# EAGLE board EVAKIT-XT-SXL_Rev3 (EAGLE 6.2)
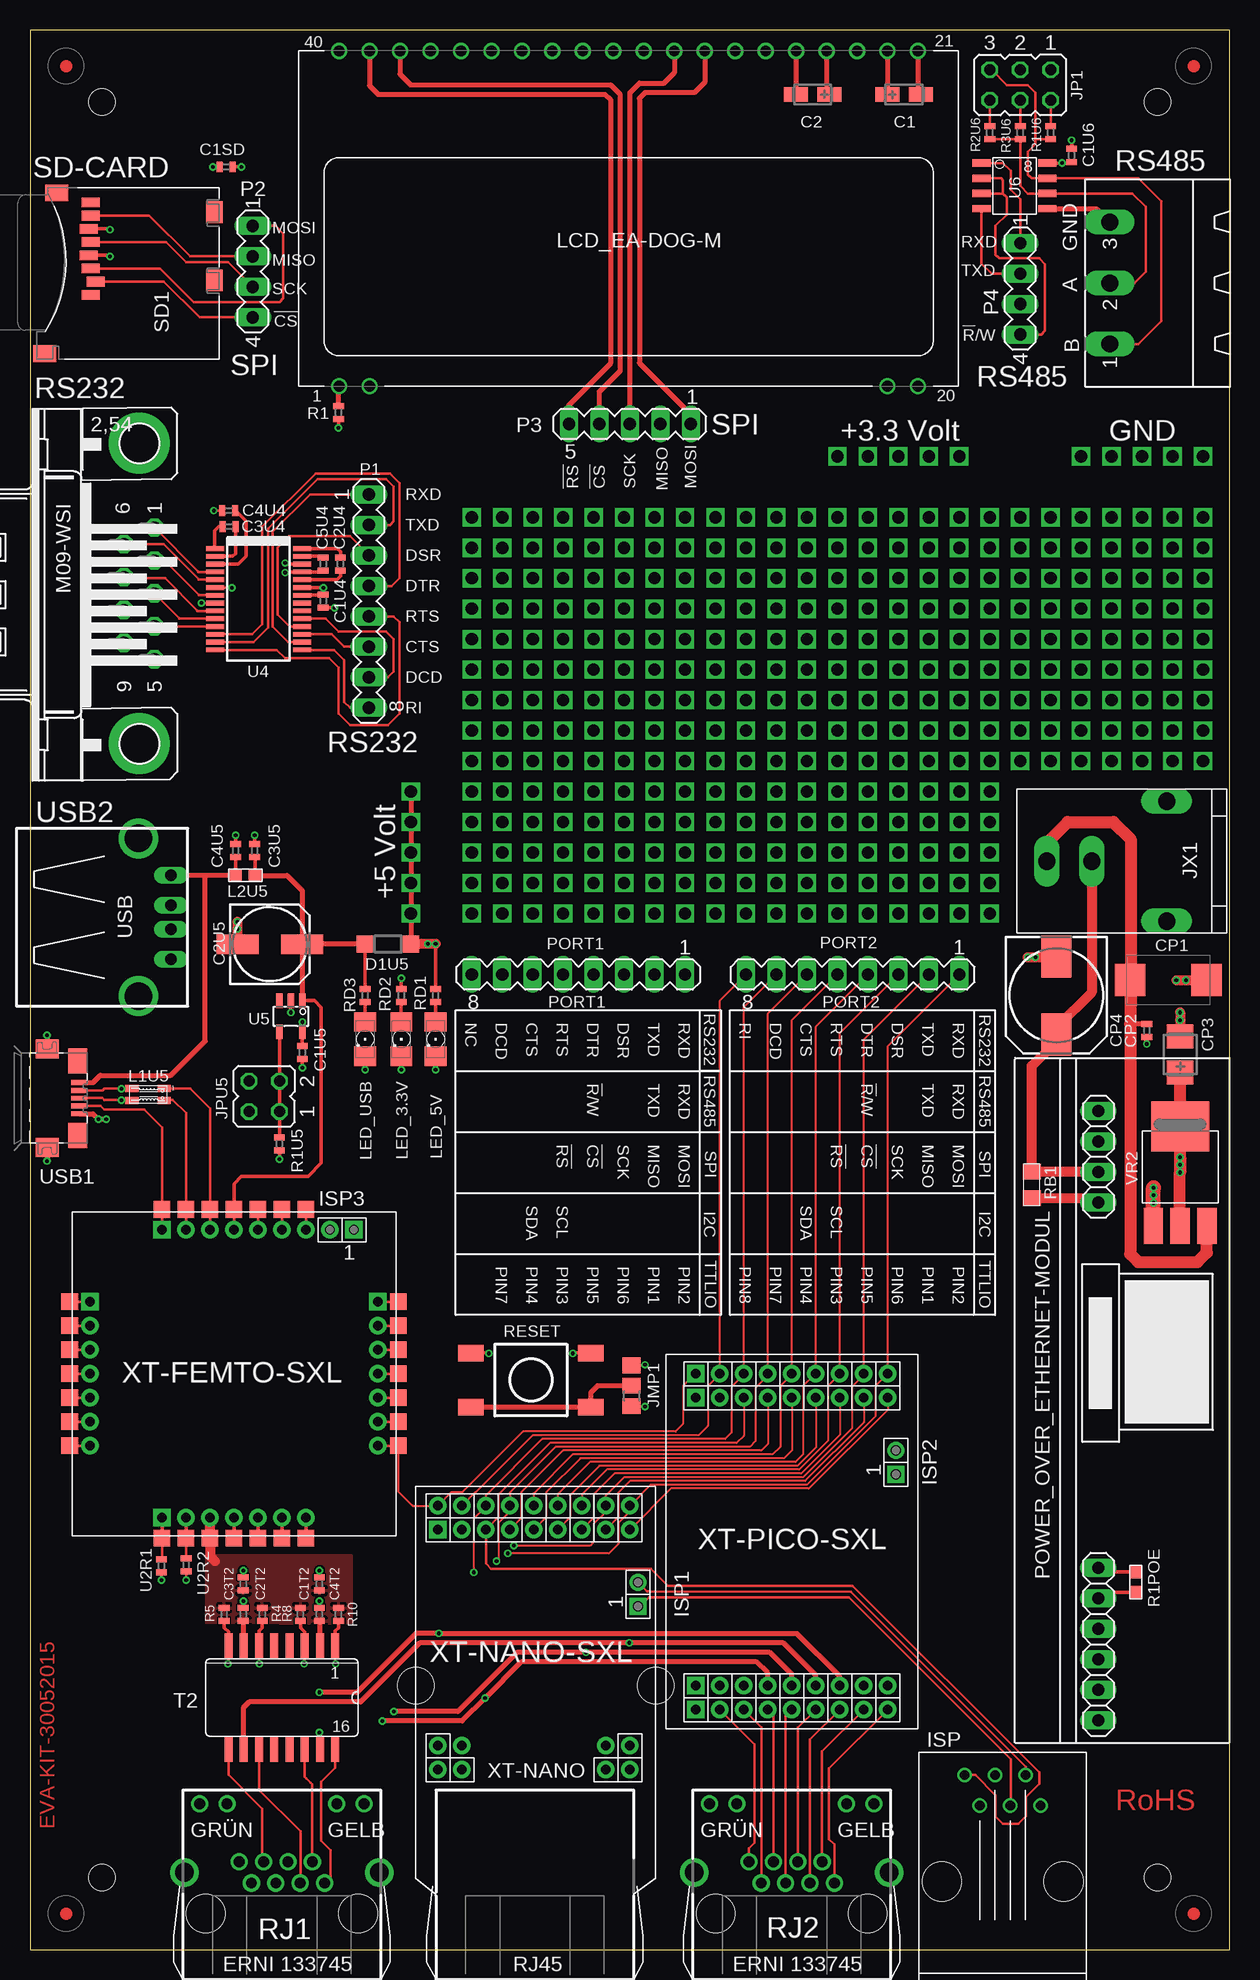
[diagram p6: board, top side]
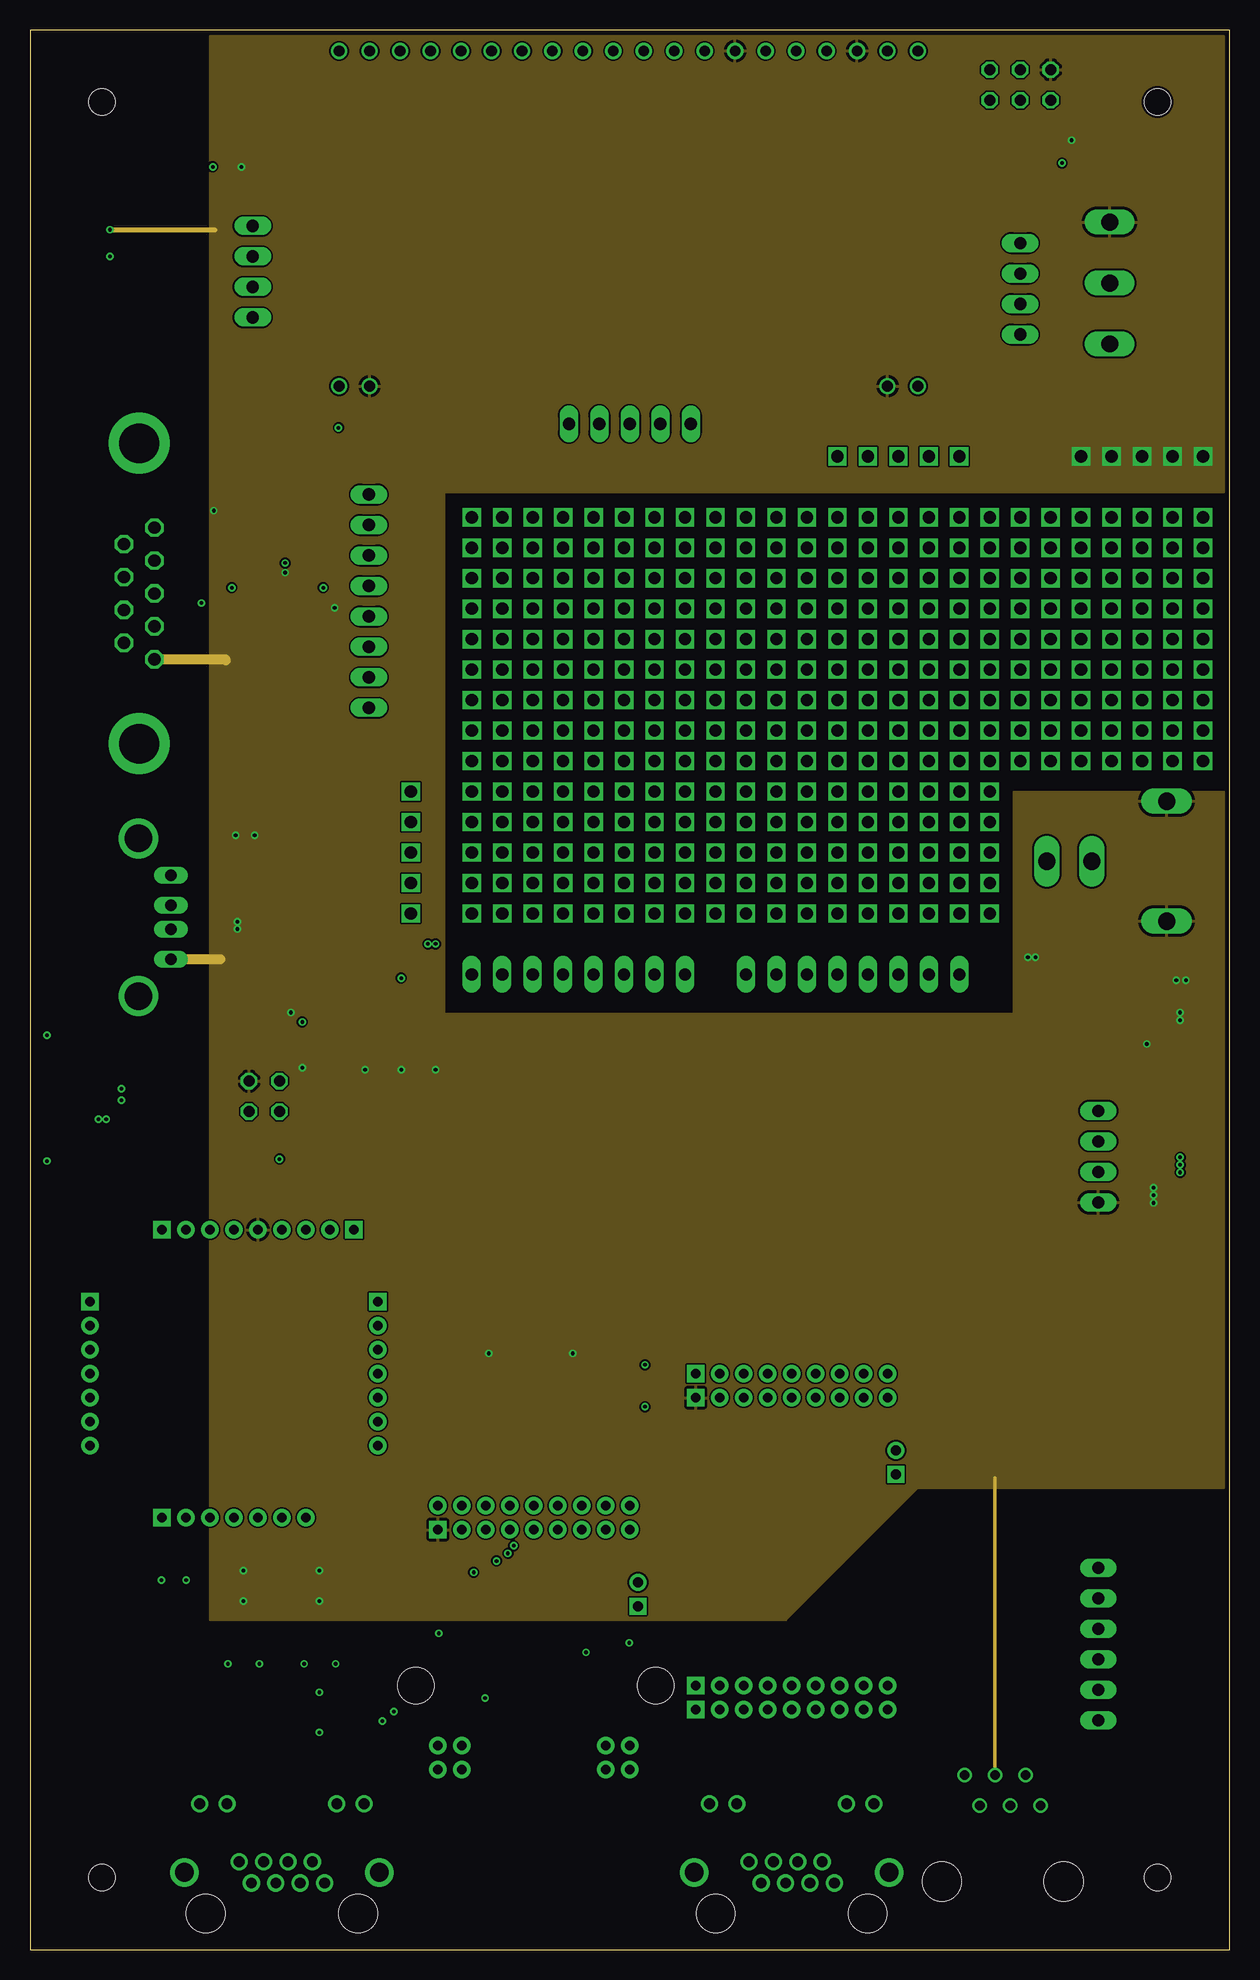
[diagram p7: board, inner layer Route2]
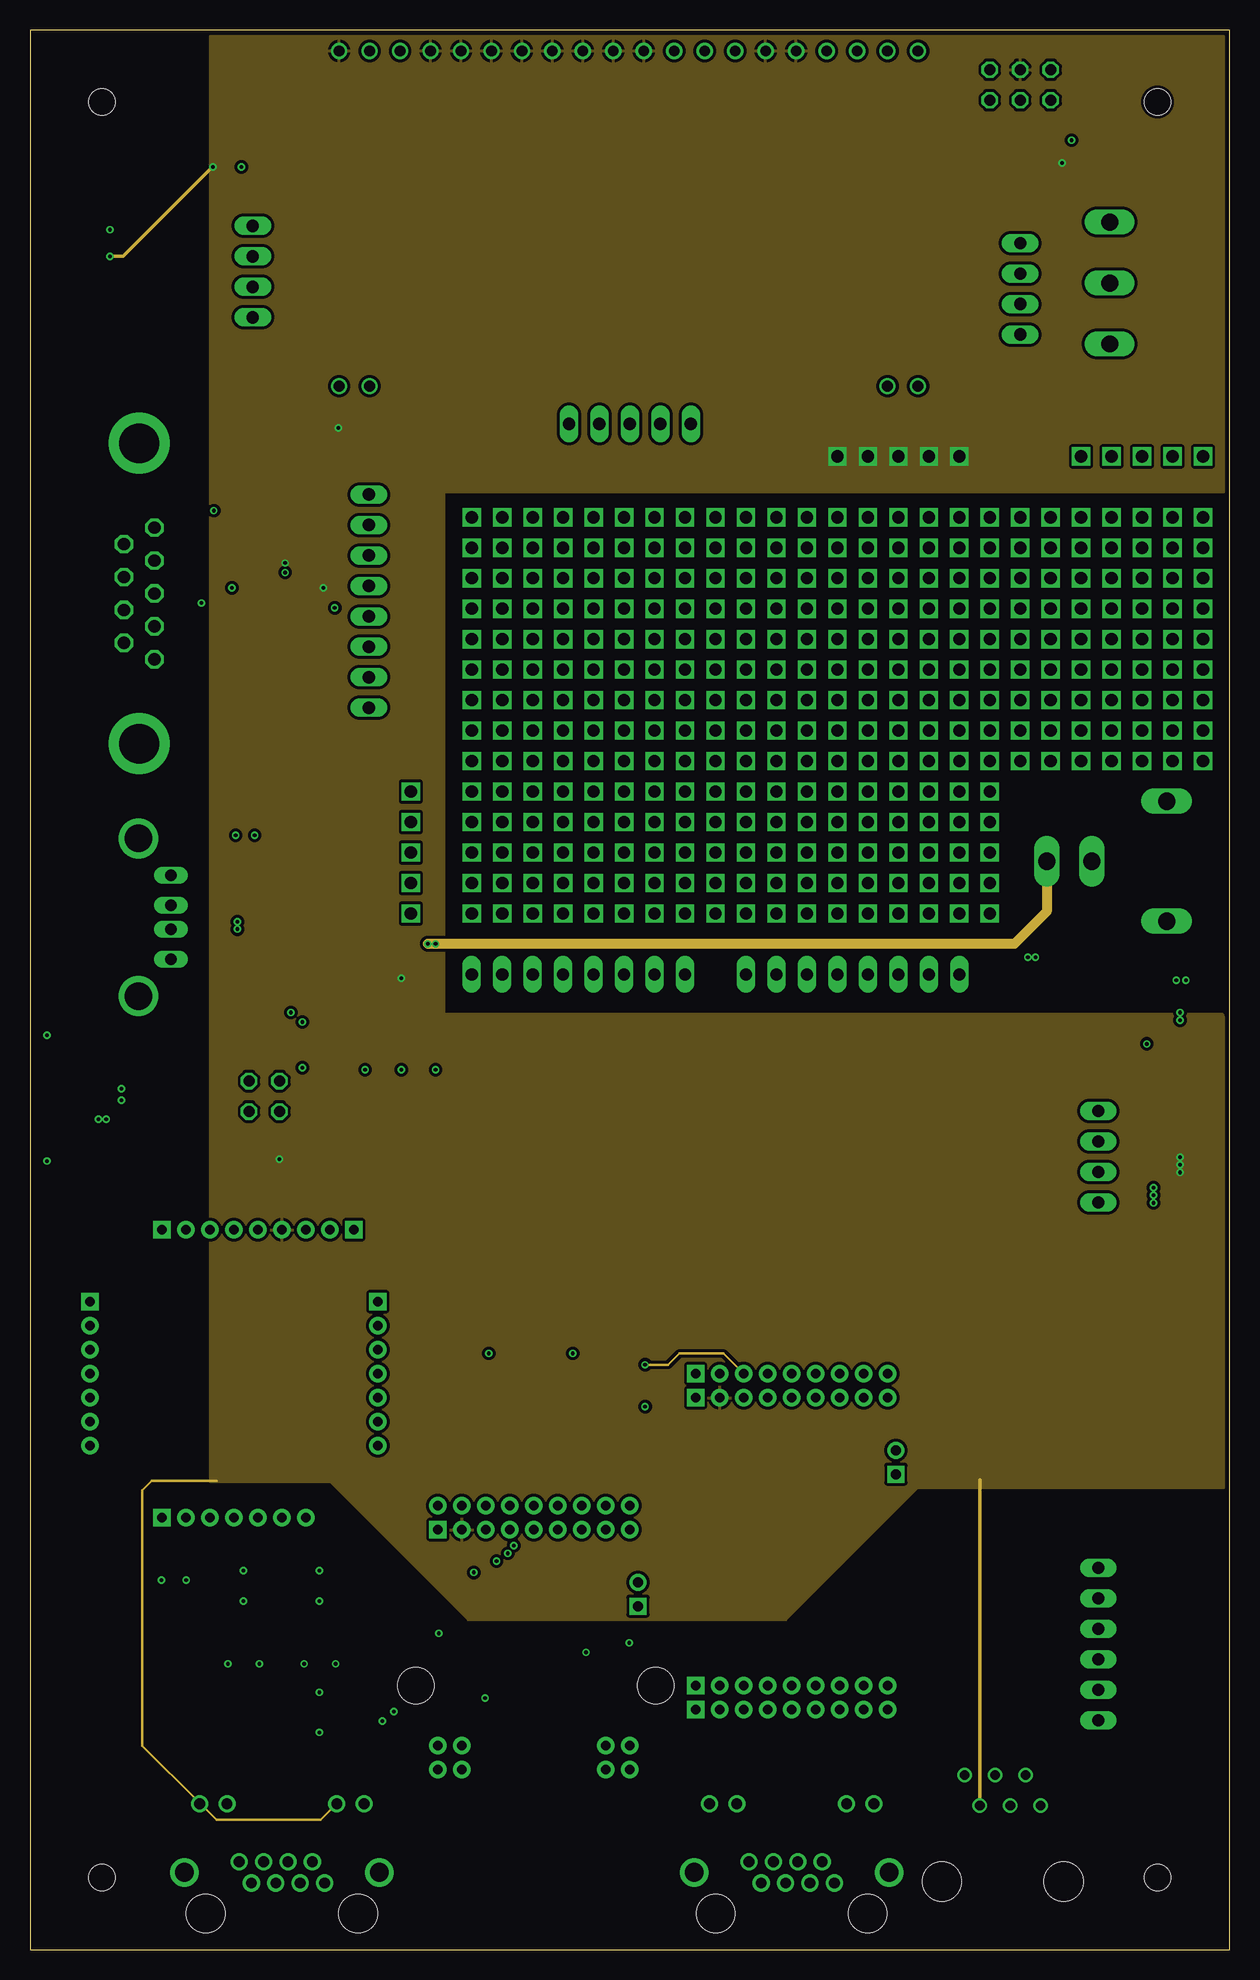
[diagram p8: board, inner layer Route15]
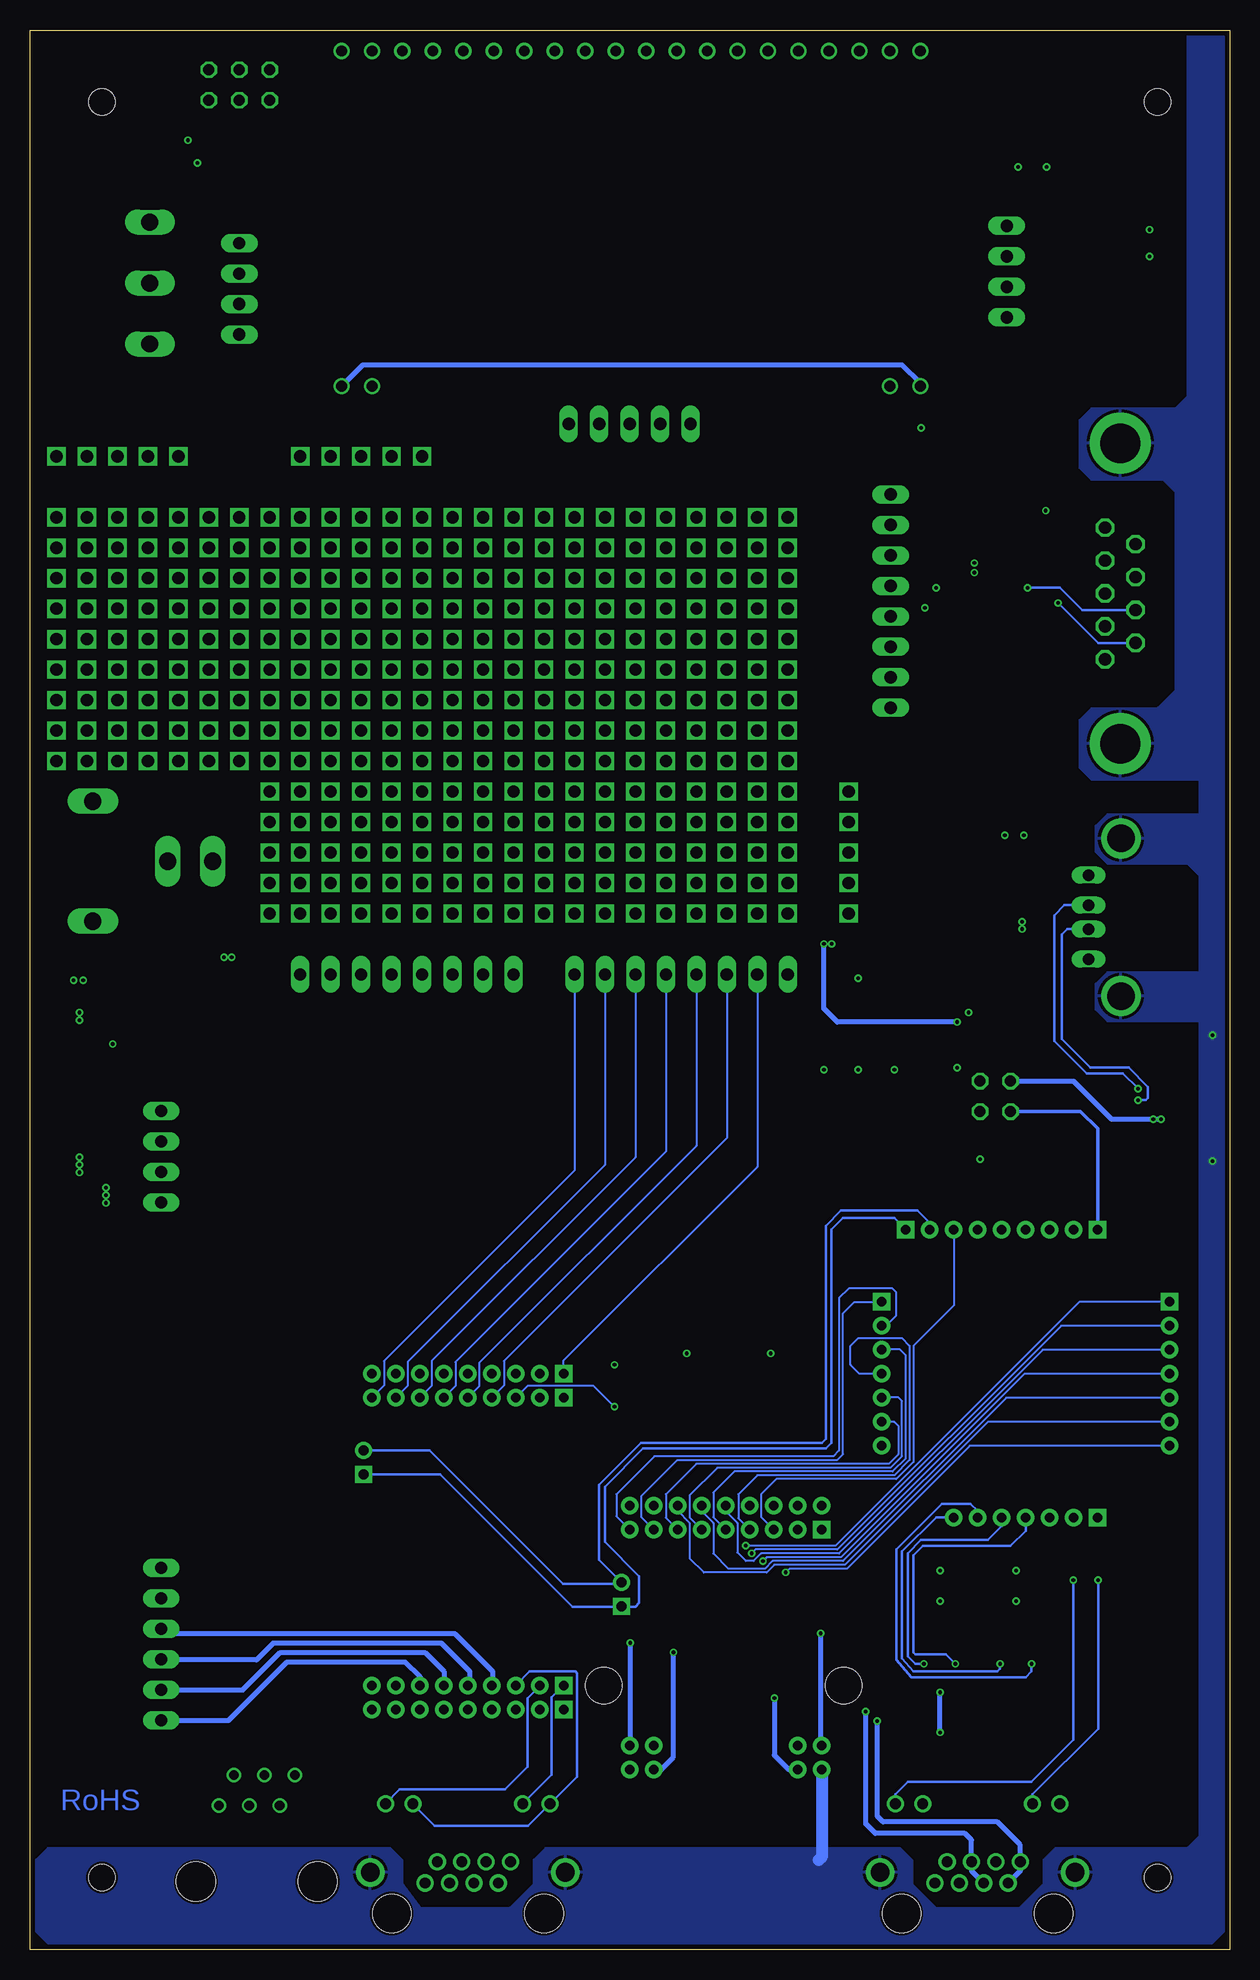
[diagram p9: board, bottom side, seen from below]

Size 100 x 160 mm. Coordinates in mm from the lower left corner, seen from the top.
Outline: 0,0 100,0 100,160 0,160 0,0
Copper layers (1*2*15*16): Top 0.035mm / dielectric 0.5mm / Route2 0.035mm / dielectric 0.5mm / Route15 0.035mm / dielectric 0.5mm / Bottom 0.035mm
Design rules: minimum track width 6mil, minimum drill 12mil, track to track 6mil, track to pad 6mil, pad to pad 6mil, via to via 6mil, smd to smd 0mil, copper to edge 8mil, drill to drill 8mil, minimum pad ring 8mil, minimum via ring 5mil, stop-mask expansion 4mil, vias tented up to drill 12mil, thermal gap 10mil
Holes 2.18 mm at 6,6 94,154 6,154 94,6
Holes 3 mm at 52.16,22 32.16,22

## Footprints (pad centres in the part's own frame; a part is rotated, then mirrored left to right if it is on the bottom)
ORCAD_X_CT3216 = smd 2 x 1.2: 1 -1.4,0; 2 1.4,0
AK0402 = smd 0.5 x 0.9: 1 -0.548,0; 2 0.548,0
153CLV-0605 = smd 3.5 x 1.6: + 2.7,0; - -2.7,0
D/7343-31R = smd 2.55 x 2.7: + 3.175,0; - -3.175,0
ORCAD_X_CT3528 = smd 2 x 2.2: 1 -1.5,0; 2 1.5,0
150CLZ-0810 = smd 3.5 x 2.5: + 3.25,0; - -3.25,0
SOD123 = smd 1.4 x 1.4: A 1.9,0; C -1.9,0
RJ12 = drill 0.8: 1 -8.89,-3.175; 2 -6.35,-1.905; 3 -8.89,-0.635; 4 -6.35,0.635; 5 -8.89,1.905; 6 -6.35,3.175 | hole 3.25: 0,-5.08; 0,5.08
ROLF_SQW1X2 = drill 0.813 pad 1.422 square: 1 0,0 | drill 0.813 pad 1.422: 2 2,0
A0R-JMP = smd 1.5 x 1.3: 1 0,1.7; 2 0,0; 3 0,-1.7
JP3Q = drill 0.914 octagon: 1 -2.54,-1.27; 2 -2.54,1.27; 3 0,-1.27; 4 0,1.27; 5 2.54,-1.27; 6 2.54,1.27
JP2Q = drill 0.914 octagon: 1 -1.27,-1.27; 2 -1.27,1.27; 3 1.27,-1.27; 4 1.27,1.27
ORCAD_X_ROKA1 = drill 1.422 pad 1.905 long: 1 0,10; 2 0,6.25; 3 -5,0; 4 5,0
2L1206 = smd 1.1 x 0.6: 1 -1.35,-0.5; 2 1.35,-0.5; 3 1.35,0.5; 4 -1.35,0.5
SMD-0603 = smd 1.1 x 1: 1 -0.85,0; 2 0.85,0
EADOGM = drill 0.9: 1 -24.13,-13.97; 2 -21.59,-13.97; 19 21.59,-13.97; 20 24.13,-13.97; 21 24.13,13.97; 22 21.59,13.97; 23 19.05,13.97; 24 16.51,13.97; 25 13.97,13.97; 26 11.43,13.97; 27 8.89,13.97; 28 6.35,13.97; 29 3.81,13.97; 30 1.27,13.97; 31 -1.27,13.97; 32 -3.81,13.97; 33 -6.35,13.97; 34 -8.89,13.97; 35 -11.43,13.97; 36 -13.97,13.97; 37 -16.51,13.97; 38 -19.05,13.97; 39 -21.59,13.97; 40 -24.13,13.97
1206 = smd 1.6 x 1.803: A -1.422,0; C 1.422,0
XT-FEMTO-SXL-PAD = smd 1.4 x 1.4: P1_0 13.7,6; P1_1 13.7,4; P1_2 13.7,2; P1_3 13.7,0; P1_4 13.7,-2; P1_5 13.7,-4; P1_6 13.7,-6; P2_0 -6,-13.7; P2_1 -4,-13.7; P2_2 -2,-13.7; P2_3 0,-13.7; P2_4 2,-13.7; P2_5 4,-13.7; P2_6 6,-13.7; P3_0 -13.7,6; P3_1 -13.7,4; P3_2 -13.7,2; P3_3 -13.7,0; P3_4 -13.7,-2; P3_5 -13.7,-4; P3_6 -13.7,-6; P4_0 -6,13.7; P4_1 -4,13.7; P4_2 -2,13.7; P4_3 0,13.7; P4_4 2,13.7; P4_5 4,13.7; P4_6 6,13.7
MA08-1 = drill 1.016 long: 1 -8.89,0; 2 -6.35,0; 3 -3.81,0; 4 -1.27,0; 5 1.27,0; 6 3.81,0; 7 6.35,0; 8 8.89,0
MA04-1 = drill 1.016 long: 1 -3.81,0; 2 -1.27,0; 3 1.27,0; 4 3.81,0
MA05-1 = drill 1.016 long: 1 -5.08,0; 2 -2.54,0; 3 0,0; 4 2.54,0; 5 5.08,0
POE_AG9000 = drill 1.016 long: 1 -26.67,0; 2 -24.13,0; 3 -21.59,0; 4 -19.05,0; 5 -16.51,0; 6 -13.97,0; 7 16.51,0; 8 19.05,0; 9 21.59,0; 10 24.13,0
SMD-0805 = smd 1.3 x 1.5: 1 -1.104,0; 2 1.104,0
LSH = smd 2.1 x 1.4: 1 -5,-2.25; 2 5,-2.25; 3 -5,2.25; 4 5,2.25
ORCAD_X_ERNI_RJ45_LED = drill 0.889 pad 1.422: 1 3.556,2.54; 2 2.54,4.318; 3 1.524,2.54; 4 0.508,4.318; 5 -0.508,2.54; 6 -1.524,4.318; 7 -2.54,2.54; 8 -3.556,4.318; A1 4.572,9.144; A2 -6.858,9.144; K1 6.858,9.144; K2 -4.572,9.144 | drill 1.575 pad 2.184: 9 8.128,3.429; 10 -8.128,3.429 | hole 3.2: 6.35,0; -6.35,0
SUBD-M09HP-WSI = drill 1.016 octagon: 1 -5.486,1.17; 2 -2.743,1.17; 3 0,1.17; 4 2.743,1.17; 5 5.486,1.17; 6 -4.115,-1.37; 7 -1.372,-1.37; 8 1.372,-1.37; 9 4.115,-1.37 | drill 3.302 pad 5.08: G1 -12.522,-0.1; G2 12.522,-0.1
MSTBA3 = drill 1.397 long: 1 -5.08,5.08; 2 0,5.08; 3 5.08,5.08
MICROSD_MICROSD = smd 0.8 x 1.5: 1 -1.94,2.7; 2 -0.84,2.3; 3 0.26,2.7; 4 1.36,2.9; 5 2.46,2.7; 6 3.56,2.9; 7 4.66,2.7; 8 5.76,2.7 | smd 1.4 x 1.9: S1 -6.85,6.55; S2 6.55,5.55 | smd 1.8 x 1.4: S3 -0.75,-7.6; S4 4.95,-7.6
SOTRANSF = smd 0.66 x 2.032: 1 -4.445,-4.343; 2 -3.175,-4.343; 3 -1.905,-4.343; 4 -0.635,-4.343; 5 0.635,-4.343; 6 1.905,-4.343; 7 3.175,-4.343; 8 4.445,-4.343; 9 4.445,4.343; 10 3.175,4.343; 11 1.905,4.343; 12 0.635,4.343; 13 -0.635,4.343; 14 -1.905,4.343; 15 -3.175,4.343; 16 -4.445,4.343
SSOP28 = smd 0.4 x 1.5: 1 -4.225,-3.625; 2 -3.575,-3.625; 3 -2.925,-3.625; 4 -2.275,-3.625; 5 -1.625,-3.625; 6 -0.975,-3.625; 7 -0.325,-3.625; 8 0.325,-3.625; 9 0.975,-3.625; 10 1.625,-3.625; 11 2.275,-3.625; 12 2.925,-3.625; 13 3.575,-3.625; 14 4.225,-3.625; 15 4.225,3.625; 16 3.575,3.625; 17 2.925,3.625; 18 2.275,3.625; 19 1.625,3.625; 20 0.975,3.625; 21 0.325,3.625; 22 -0.325,3.625; 23 -0.975,3.625; 24 -1.625,3.625; 25 -2.275,3.625; 26 -2.925,3.625; 27 -3.575,3.625; 28 -4.225,3.625
SOT23-5 = smd 0.55 x 1.2: 1 -0.95,-1.3; 2 0,-1.3; 3 0.95,-1.3; 4 0.95,1.3; 5 -0.95,1.3
SO-8 = smd 0.61 x 1.524: 1 -1.905,-2.743; 2 -0.635,-2.743; 3 0.635,-2.743; 4 1.905,-2.743; 5 1.905,2.743; 6 0.635,2.743; 7 -0.635,2.743; 8 -1.905,2.743
ZX62R-AB-5P(11) = smd 1.35 x 0.4: 1 2.675,1.3; 2 2.675,0.65; 3 2.675,0; 4 2.675,-0.65; 5 2.675,-1.3 | smd 1.9 x 1.6: M1 0,-4.1; M2 0,4.1 | smd 1.6 x 2.1: M3 2.55,3.1; M4 2.55,-3.1
USB_A_1 = drill 2.3 pad 3: G1 -6.57,0; G2 6.57,0 | drill 0.95 long: P1 -3.5,2.71; P2 -1,2.71; P3 1,2.71; P4 3.5,2.71
DPAK_223 = smd 1.6 x 2.997: 1 -2.235,-4.134; 2 -0.013,-4.134; 3 2.235,-4.134 | smd 4.826 x 4.191: 4 0,4.146
XT-FEMTO-SXL-PIN = drill 0.813 pad 1.422 square: P1_0 12,6; P2_0 -6,-12; P3_0 -12,6; P4_0 -6,12 | drill 0.813 pad 1.422: P1_1 12,4; P1_2 12,2; P1_3 12,0; P1_4 12,-2; P1_5 12,-4; P1_6 12,-6; P2_1 -4,-12; P2_2 -2,-12; P2_3 0,-12; P2_4 2,-12; P2_5 4,-12; P2_6 6,-12; P3_1 -12,4; P3_2 -12,2; P3_3 -12,0; P3_4 -12,-2; P3_5 -12,-4; P3_6 -12,-6; P4_1 -4,12; P4_2 -2,12; P4_3 0,12; P4_4 2,12; P4_5 4,12; P4_6 6,12
XT-NANO-XXL/SXL = drill 0.813 pad 1.422: FLASH 8,-10; P1_2 -6,10; P1_3 -4,10; P1_4 -2,10; P1_5 0,10; P1_6 2,10; P1_7 4,10; P1_8 6,10; P1_9 8,10; P2_1 -8,12; P2_2 -6,12; P2_3 -4,12; P2_4 -2,12; P2_5 0,12; P2_6 2,12; P2_7 4,12; P2_8 6,12; P2_9 8,12; POE12 -8,-8; POE36 8,-8; POE45 6,-10; POE78 -6,-10; SHIELD -8,-10 | drill 0.813 pad 1.422 square: P1_1 -8,10
XT-PICO-XXL/SXL = drill 0.813 pad 1.422 square: P1_1 -8,12; P2_1 -8,14; P3_1 -8,-12; P4_1 -8,-14 | drill 0.813 pad 1.422: P1_2 -6,12; P1_3 -4,12; P1_4 -2,12; P1_5 0,12; P1_6 2,12; P1_7 4,12; P1_8 6,12; P1_9 8,12; P2_2 -6,14; P2_3 -4,14; P2_4 -2,14; P2_5 0,14; P2_6 2,14; P2_7 4,14; P2_8 6,14; P2_9 8,14; P3_2 -6,-12; P3_3 -4,-12; P3_4 -2,-12; P3_5 0,-12; P3_6 2,-12; P3_7 4,-12; P3_8 6,-12; P3_9 8,-12; P4_2 -6,-14; P4_3 -4,-14; P4_4 -2,-14; P4_5 0,-14; P4_6 2,-14; P4_7 4,-14; P4_8 6,-14; P4_9 8,-14

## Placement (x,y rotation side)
C1  1uF 16V SizeA  [ORCAD_X_CT3216]  72.87,154.62 0 top
C1SD  100nF  [AK0402]  16.35,148.59 180 top
C1T2  100nF  [AK0402]  24.13,27.94 90 top
C1U4  100nF  [AK0402]  24.45,112.39 270 top
C1U5  100nF  [AK0402]  22.7,74.77 270 top
C1U6  100nF  [AK0402]  86.84,149.54 270 top
C2  2.2uF 6V SizeA  [ORCAD_X_CT3216]  65.25,154.62 180 top
C2T2  100nF  [AK0402]  17.78,27.94 270 top
C2U4  100nF  [AK0402]  25.88,115.49 90 top
C2U5  100uF 16V RM3.5mm  [153CLV-0605]  20,83.8 0 top
C3T2  100nF  [AK0402]  17.78,30.48 90 top
C3U4  100nF  [AK0402]  16.59,118.6 180 top
C3U5  100nF  [AK0402]  18.73,91.6 270 top
C4T2  100nF  [AK0402]  24.13,30.48 270 top
C4U4  100nF  [AK0402]  16.57,119.94 180 top
C4U5  100nF  [AK0402]  17.14,91.6 270 top
C5U4  100nF  [AK0402]  24.45,115.49 270 top
CP1  10uF 35V SizeD  [D/7343-31R]  94.9,80.82 180 top
CP2  10nF  [AK0402]  93.11,76.6 90 top
CP3  10uF 10V SizeB  [ORCAD_X_CT3528]  95.88,74.61 90 top
CP4  470uF 10V 3.5 x 8  [150CLZ-0810]  85.57,79.53 270 top
D1U5  MBR0520LT1G  [SOD123]  29.84,83.82 180 top
ISP  RJ12  [RJ12]  81.09,5.66 270 top
ISP1  [ROLF_SQW1X2]  50.69,28.61 90 top
ISP2  [ROLF_SQW1X2]  72.19,39.61 90 top
ISP3  [ROLF_SQW1X2]  27,60 180 top
JMP1  0R-JUMPA  [A0R-JMP]  50.16,46.99 180 top
JP1  PIN 3x2x2.54  [JP3Q]  82.55,155.42 180 top
JPU5  PIN 2x2x2.54  [JP2Q]  19.53,71.12 90 top
JX1  ROCA_BUCHSE_DIN45323  [ORCAD_X_ROKA1]  94.76,90.71 90 top
L1U5  Würth 744232090  [2L1206]  9.84,71.28 180 top
L2U5  Würth 742792601  [SMD-0603]  17.94,89.53 180 top
LCD_EA-DOG-M  EADOGM  [EADOGM]  49.9,144.28 0 top
LED_3.3V  KPTD-3216MGCK Grün  [1206]  30.96,75.88 270 top
LED_5V  KPTD-3216MGCK Grün  [1206]  33.81,75.88 270 top
LED_USB  KPTD-3216MGCK Grün  [1206]  27.94,75.88 270 top
M1  XT-FEMTO-SXL2  [XT-FEMTO-SXL-PAD]  17,48 0 top
MA1  [MARKER_RUND]  97,3 0 top
MA2  [MARKER_RUND]  3,157 0 top
MA3  [MARKER_RUND]  97,157 0 top
MA4  [MARKER_RUND]  3,3 0 top
P1  PIN 8x1x2.54  [MA08-1]  28.26,112.39 270 top
P2  PIN 4x1x2.54  [MA04-1]  18.57,139.86 270 top
P3  PIN 5x1x2.54  [MA05-1]  50.01,127.16 180 top
P4  PIN 4x1x2.54  [MA04-1]  82.55,138.43 270 top
PORT1  PIN 8x1x2.54  [MA08-1]  45.72,81.28 180 top
PORT2  PIN 8x1x2.54  [MA08-1]  68.58,81.28 180 top
POWER_OVER_ETHERNET-MODUL  AG9050-S  [POE_AG9000]  89.07,45.77 90 top
R1  15R  [AK0402]  25.72,128.11 90 top
R1POE  383R  [SMD-0603]  92.18,30.63 90 top
R1U5  100K  [AK0402]  20.8,67.15 90 top
R1U6  560R  [AK0402]  85.09,151.45 270 top
R2U6  120R  [AK0402]  80.01,151.45 270 top
R3U6  560R  [AK0402]  82.55,151.45 270 top
R4  49R9  [AK0402]  19.37,27.94 90 top
R5  49R9  [AK0402]  16.19,27.94 90 top
R8  49R9  [AK0402]  22.54,27.94 90 top
R10  49R9  [AK0402]  25.72,27.94 90 top
RB1  240R 0,25W  [SMD-0805]  83.5,63.74 270 top
RD1  1K  [AK0402]  33.81,79.53 90 top
RD2  330R  [AK0402]  30.96,79.53 90 top
RD3  330R  [AK0402]  27.94,79.53 270 top
RESET  LSH  [LSH]  41.75,47.47 180 top
RJ1  KYCON GWL-S9-88-G-Y  [ORCAD_X_ERNI_RJ45_LED]  21,3 0 top
RJ2  KYCON GWL-S9-88-G-Y  [ORCAD_X_ERNI_RJ45_LED]  63.5,3 0 top
RS232  SUBD_M+F09WSI-MALE  [SUBD-M09HP-WSI]  9.21,113.03 270 top
RS485  5.08/03/90G 3.2SN BK BX  [MSTBA3]  95.09,138.91 90 top
SD1  MICROSD_SF-MICROSD  [MICROSD_MICROSD]  7.78,139.86 90 top
T2  Würth 749013011A  [SOTRANSF]  21,21 180 top
U2R1  330R  [AK0402]  10.95,31.99 90 top
U2R2  330R  [AK0402]  13.02,32.07 90 top
U4  MAX3243EAI  [SSOP28]  19.05,112.55 270 top
U5  TPS2041B  [SOT23-5]  21.75,77.79 180 top
U6  MAX3072E  [SO-8]  82.07,147 270 top
U$7  [ROLF_LOGOBL]  not placed on the board
USB1  ZX62R-AB-5P(11)A  [ZX62R-AB-5P(11)]  1.43,70.96 0 top
USB2  Lumberg 2410 02  [USB_A_1]  9.05,86.04 270 top
VR2  LT1086CM-3.3  [DPAK_223]  95.89,64.45 0 top
XT-FEMTO-SXL  XT-FEMTO-SXL1  [XT-FEMTO-SXL-PIN]  17,48 0 top
XT-NANO-SXL  X-TNANO-XXL/SXL  [XT-NANO-XXL/SXL]  42,25 0 top
XT-PICO-SXL  XT-PICO-XXL/SXL  [XT-PICO-XXL/SXL]  63.5,34 0 top

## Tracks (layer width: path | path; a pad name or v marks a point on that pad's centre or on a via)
#RESET  (via drill 0.3 pad 0.61)
  Top 0.152: XT-PICO-SXL.P1_3 59.5,42.83 58.9,42.23 43.34,42.23 39.05,37.94 39.05,36.05 XT-NANO-SXL.P1_3
  Top 0.203: XT-FEMTO-SXL.P4_6 M1.P4_6 | ISP.1 78.8,14.55 80.49,12.86 80.49,11.11 81.12,10.48 82.39,10.48 83.03,11.11 83.03,12.7 84.14,13.81 84.14,14.76 68.58,30.32 53.18,30.32 51.75,31.75 38.42,31.75 38,32.17 XT-NANO-SXL.P1_3 | JMP1.1 51.23,45.29 v51.28,45.24
  Bottom 0.152: XT-FEMTO-SXL.P4_6 23,53.68 26.35,50.32 26.35,40.64 27.78,39.21 37.78,39.21 39.05,37.94 39.05,36.05 XT-NANO-SXL.P1_3 | XT-PICO-SXL.P1_3 58.51,46.99 53.02,46.99 v51.28,45.24
+3.3V  (via drill 0.3 pad 0.61, 1.02)
  Top 0.203: M1.P4_5 XT-FEMTO-SXL.P4_5
  Top 0.305: U4.22 24.38,112.88 C1U4.1 v24.45,113.51 24.43,113.53 U4.23 | U4.26 21.36,115.48 v21.27,115.57 | v20.8,65.88 R1U5.1 | RD2.2 v30.96,80.96 | SD1.4 6.67,141.22 v6.67,141.13 | C1SD.2 v15.24,148.59 | R1.1 v25.72,126.84 | U6.8 v86.04,148.91 86.75,148.91 C1U6.2
  Top 0.406: LCD_EA-DOG-M.25 63.87,154.65 C2.2
  Top 1.016: 95.73,73.11 CP3.1 | 95.73,60.33 VR2.2 95.87,64.76 v95.89,64.77 | v95.89,66.04 v95.89,64.77 | v95.89,64.77 VR2.4 | VR2.4 | VR2.4 CP3.1 | CP3.1
  Route15 0.203: 15.56,39.05 10.16,39.05 9.37,38.26 9.37,16.99 14.14,12.21 RJ1.A2 14.21,12.14 15.56,10.79 24.22,10.79 RJ1.A1
  Route15 0.305: v6.67,141.13 7.78,141.13 v15.24,148.59 | ISP.2 79.19,38.69 79.18,39.16
  other vias: 95.89,65.41 67.31,124.46 69.85,124.46 72.39,124.46 74.93,124.46 77.47,124.46
  pour Route15 (isolate 0.254): 99.5,38.5 74,38.5 63,27.5 36.5,27.5 25,39 15,39 15,159.5 99.5,159.5 99.5,121.5 34.5,121.5 34.5,78 99.25,78 arc-90 99.5,77.75
+5V  (via drill 0.3 pad 0.61, 1.02)
  Top 0.305: U5.5 C1U5.1 | RD1.2 v33.81,83.82
  Top 0.406: 91.72,77.15 91.8,77.23 91.89,77.14 CP2.2 | U5.5 v22.7,77.31 | v31.75,96.52 v31.75,93.98 v31.75,91.44 v31.75,88.9 v31.75,86.36 D1U5.C
  Top 0.813: D1U5.C v33.18,83.82 v33.81,83.82
  Top 1.016: JX1.1 84.75,92.22 86.52,93.98 90.33,93.98 91.76,92.55 91.76,78.63 CP1.+ 91.72,77.15 91.72,57.98 92.39,57.31 97.31,57.31 98.11,58.1 98.11,60.31 VR2.3
  Route15 0.813: JX1.1 84.75,86.5 82.07,83.82 v33.81,83.82 v33.18,83.82
  Bottom 0.406: v22.7,77.31 32.7,77.31 33.81,78.42 v33.81,83.82
AVDD
  Top 0.406: T2.7 17.82,27.35 C2T2.2 | T2.2 24.18,27.35 C1T2.1
  Top 0.813: XT-FEMTO-SXL.P2_2 M1.P2_2 15,32.78 15.4,32.38
  pour Top: 14.68,32.86 26.8,32.86 26.8,27.15 14.68,27.23
CP1
  Top 0.305: R1POE.1 89.59,29.78 POWER_OVER_ETHERNET-MODUL.5
CP2
  Top 0.305: R1POE.2 89.39,31.48 POWER_OVER_ETHERNET-MODUL.6
DM  (via drill 0.3 pad 0.61)
  Top 0.203: USB1.2 6.05,71.61 6.19,71.75 v7.62,71.75 8.47,71.75 L1U5.2
  Bottom 0.203: USB2.P2 13.76,87.04 14.61,86.2 14.61,75.72 11.91,73.03 8.89,73.03 v7.62,71.75
DP  (via drill 0.3 pad 0.61)
  Top 0.203: USB1.3 6.03,70.96 6.19,70.8 v7.62,70.8 8.47,70.8 L1U5.3
  Bottom 0.203: USB2.P3 13.54,85.04 13.97,84.61 13.97,75.88 11.59,73.5 8.41,73.5 6.83,71.91 6.83,70.96 6.99,70.8 v7.62,70.8
DP_SPI_CLK
  Top 0.406: P3.3 50.01,154.78 50.8,155.57 52.86,155.57 53.71,156.42 LCD_EA-DOG-M.29
DP_SPI_CS
  Top 0.406: P3.4 47.47,129.86 49.21,131.6 49.21,154.62 48.42,155.42 31.75,155.42 30.85,156.32 LCD_EA-DOG-M.38
DP_SPI_MOSI
  Top 0.406: LCD_EA-DOG-M.28 56.25,155.63 55.4,154.78 51.28,154.78 50.8,154.31 50.8,132.24 55.09,127.95 P3.1
DP_SPI_RS
  Top 0.406: P3.5 44.93,128.75 48.42,132.24 48.42,154.15 47.94,154.62 29.05,154.62 28.31,155.36 LCD_EA-DOG-M.39
E1  (via drill 0.81 pad 1.42)
  other vias: 36,17
E2  (via drill 0.81 pad 1.42)
  other vias: 48,17
GND  (via drill 0.3 pad 0.61, 1.02)
  Top 0.203: C1T2.2 v24.13,29.05 | C2T2.1 v17.78,29.05 | C3T2.2 v17.78,31.59 | v24.13,31.59 C4T2.1 | XT-FEMTO-SXL.P4_4 M1.P4_4 | C4U4.2 v15.32,119.94
  Top 0.305: C5U4.2 24.41,114.83 U4.25 21.32,114.83 v21.27,114.78 | C1U4.2 v25.39,111.85 v25.4,111.84 | v17.14,92.87 C4U5.1 | v18.73,92.87 C3U5.1 | U5.2 v21.75,78.11 | C1U5.2 v22.7,73.5 | LED_USB.C v27.94,73.34 | LED_3.3V.C v30.96,73.34 | LED_5V.C v33.81,73.34 | SD1.6 6.67,143.42 v6.67,143.35 | C1SD.1 v17.62,148.59 | RESET.2 38.23,49.72 v38.26,49.69 | RESET.1 45.27,49.72 v45.24,49.69 | v86.84,150.81 C1U6.1
  Top 0.406: v93.11,75.49 93.11,75.41 CP2.1 | USB1.5 5.27,69.66 v5.71,69.22 v6.35,69.22 | U6.5 88.9,145.1 RS485.3
  Top 0.813: RB1.2 88.72,62.63 POWER_OVER_ETHERNET-MODUL.7 | v95.89,78.11 v95.89,77.47 95.89,76.27 CP3.2 | v95.57,80.8 v96.36,80.8 97.9,80.8 CP1.- | C2U5.- v17.3,85.66 | v83.19,82.71 85.49,82.71 CP4.-
  Top 1.27: VR2.1 93.65,63.49 v93.66,63.5
  Route2 0.305: ISP.3 80.45,39.3
  Route2 0.406: v6.67,143.35 15.4,143.35
  Route2 0.813: USB2.P4 15.87,82.54 15.88,82.55 | RS232.5 16.28,107.54 16.35,107.47
  Bottom 0.406: JPU5.4 13.02,72.39 9.84,69.22 v5.71,69.22
  other vias: 93.66,62.23 93.66,62.87 87.63,124.46 90.17,124.46 92.71,124.46 95.25,124.46 97.79,124.46 17.3,85.06 83.82,82.71
  pour Route2: 99.5,159.5 99.5,121.5 34.5,121.5 34.5,78 82,78 82,96.5 99.5,96.5 99.5,38.5 74,38.5 63,27.5 15,27.5 15,159.5 99.46,159.46
N$1
  Top 0.203: M1.P2_1 13,32.63 U2R2.2
  Top 0.305: M1.P2_1 XT-FEMTO-SXL.P2_1
N$2  (via drill 0.3 pad 0.61)
  Top 0.203: U2R1.1 v10.95,30.8
  Bottom 0.203: RJ1.K2 16.43,12.94 10.95,18.41 v10.95,30.8
N$3
  Top 0.305: U4.28 25.62,116.78 25.88,116.52 C2U4.2
N$4  (via drill 0.3 pad 0.61)
  Top 0.203: U2R2.1 v13.02,30.8
  Bottom 0.203: RJ1.K1 27.86,12.94 26.83,13.97 16.51,13.97 13.02,17.46 v13.02,30.8
N$5
  Top 0.406: R1.2 25.72,130.26 LCD_EA-DOG-M.1
  Bottom 0.406: LCD_EA-DOG-M.1 25.77,130.54 27.3,132.08 72.26,132.08 LCD_EA-DOG-M.20
N$6
  Top 0.203: M1.P2_0 11,32.58 U2R1.2
  Top 0.305: M1.P2_0 XT-FEMTO-SXL.P2_0
N$7
  Top 0.406: LCD_EA-DOG-M.24 66.41,154.86 C2.1
N$8
  Top 0.305: C3U4.2 15.73,118.6 15.4,118.27 15.4,116.81 U4.1
N$9
  Top 0.406: LCD_EA-DOG-M.21 74.03,154.86 C1.2
N$10
  Top 0.305: C3U4.1 17.14,116.36 16.91,116.13 U4.2
N$11
  Top 0.406: LCD_EA-DOG-M.22 71.49,154.65 C1.1
N$12
  Top 0.305: U4.24 25.6,114.18 25.88,114.46 C2U4.1
N$13
  Top 0.305: U4.27 24.28,116.13 C5U4.1
N$14
  Top 0.305: C4U4.1 17.14,119.94 18.02,119.06 18.02,116.13 17.37,115.48 U4.3
N$15
  Top 0.305: C4U5.2 17.14,89.59 L2U5.2
  Top 0.406: USB1.1 5.27,72.26 5.87,72.87 11.75,72.87 14.61,75.72 14.61,89.53 | 14.61,89.53 USB2.P1 | L2U5.2 14.61,89.53
N$16
  Top 0.305: U5.4 20.8,72.71 JPU5.3 JPU5.1 R1U5.2
N$17
  Top 0.203: JP1.2 R1U6.1
N$18
  Top 0.203: JP1.6 R2U6.1
N$19
  Top 0.203: JP1.4 R3U6.1
N$20
  Top 0.305: RD1.1 LED_5V.A
N$21
  Top 0.305: RD2.1 LED_3.3V.A
N$22
  Top 0.305: LED_USB.A RD3.2
N$23
  Top 0.203: RJ2.1 67.06,8.76 66.6,9.21 66.6,15.1 XT-PICO-SXL.P4_9
N$24
  Top 0.203: RJ2.2 66.04,16.54 XT-PICO-SXL.P4_8
N$25
  Top 0.203: RJ2.3 65.02,17.52 XT-PICO-SXL.P4_7
N$26
  Top 0.203: RJ2.6 61.98,19.52 XT-PICO-SXL.P4_4
N$27
  Bottom 0.203: XT-PICO-SXL.P3_2 57.5,21.96 58.51,20.95 58.51,15.24 60.41,13.34 69.17,13.34 RJ2.K1
N$28
  Bottom 0.203: XT-PICO-SXL.P3_1 55.56,22 56.52,21.03 56.52,14.55 RJ2.K2
N$29
  Bottom 0.203: RJ2.A1 68.07,12.1 66.29,10.32 58.47,10.32 RJ2.A2 54.38,14.41 54.38,23.02 54.54,23.18 58.35,23.18 59.5,22.03 XT-PICO-SXL.P3_3
N$30
  Top 0.406: RESET.4 RESET.3 46.75,46.43 47.31,46.99 JMP1.2
N$34
  Top 0.203: RJ2.4 64.01,18.51 XT-PICO-SXL.P4_6
N$35
  Top 0.203: RJ2.5 62.99,19.49 XT-PICO-SXL.P4_5
N$36
  Top 0.203: RJ2.7 60.96,18.54 XT-PICO-SXL.P4_3
N$38  (via drill 1.02)
  other vias: 80.01,96.52
N$39
  Top 0.203: RJ2.8 59.94,8.42 60.41,8.89 60.41,17.09 XT-PICO-SXL.P4_2
N$40  (via drill 1.02)
  other vias: 90.17,99.06
N$41  (via drill 1.02)
  other vias: 85.09,99.06
N$42  (via drill 1.02)
  other vias: 92.71,99.06
N$43  (via drill 1.02)
  other vias: 87.63,99.06
N$44  (via drill 1.02)
  other vias: 95.25,99.06
N$45  (via drill 1.02)
  other vias: 82.55,99.06
N$46  (via drill 1.02)
  other vias: 80.01,99.06
N$47  (via drill 1.02)
  other vias: 90.17,101.6
N$48  (via drill 1.02)
  other vias: 85.09,101.6
N$49  (via drill 1.02)
  other vias: 92.71,101.6
N$50  (via drill 1.02)
  other vias: 87.63,101.6
N$51  (via drill 1.02)
  other vias: 95.25,101.6
N$52  (via drill 1.02)
  other vias: 82.55,101.6
N$53  (via drill 1.02)
  other vias: 80.01,101.6
N$54  (via drill 1.02)
  other vias: 97.79,104.14
N$55  (via drill 1.02)
  other vias: 97.79,106.68
N$56  (via drill 1.02)
  other vias: 97.79,109.22
N$57  (via drill 1.02)
  other vias: 97.79,111.76
N$58  (via drill 1.02)
  other vias: 97.79,114.3
N$59  (via drill 1.02)
  other vias: 97.79,116.84
N$60  (via drill 1.02)
  other vias: 97.79,119.38
N$62  (via drill 1.02)
  other vias: 97.79,99.06
N$63  (via drill 1.02)
  other vias: 97.79,101.6
N$64  (via drill 1.02)
  other vias: 80.01,86.36
N$65  (via drill 1.02)
  other vias: 80.01,88.9
N$66  (via drill 1.02)
  other vias: 80.01,91.44
N$67  (via drill 1.02)
  other vias: 80.01,93.98
N$81  (via drill 1.02)
  other vias: 46.99,86.36
N$82  (via drill 1.02)
  other vias: 41.91,86.36
N$83  (via drill 1.02)
  other vias: 49.53,86.36
N$84  (via drill 1.02)
  other vias: 44.45,86.36
N$85  (via drill 1.02)
  other vias: 52.07,86.36
N$86  (via drill 1.02)
  other vias: 39.37,86.36
N$87  (via drill 1.02)
  other vias: 54.61,86.36
N$88  (via drill 1.02)
  other vias: 36.83,86.36
N$89  (via drill 1.02)
  other vias: 67.31,86.36
N$90  (via drill 1.02)
  other vias: 62.23,86.36
N$91  (via drill 1.02)
  other vias: 69.85,86.36
N$92  (via drill 1.02)
  other vias: 64.77,86.36
N$93  (via drill 1.02)
  other vias: 72.39,86.36
N$94  (via drill 1.02)
  other vias: 59.69,86.36
N$95  (via drill 1.02)
  other vias: 74.93,86.36
N$96  (via drill 1.02)
  other vias: 57.15,86.36
N$97  (via drill 1.02)
  other vias: 46.99,88.9
N$98  (via drill 1.02)
  other vias: 41.91,88.9
N$99  (via drill 1.02)
  other vias: 49.53,88.9
N$100  (via drill 1.02)
  other vias: 44.45,88.9
N$101  (via drill 1.02)
  other vias: 52.07,88.9
N$102  (via drill 1.02)
  other vias: 39.37,88.9
N$103  (via drill 1.02)
  other vias: 54.61,88.9
N$104  (via drill 1.02)
  other vias: 36.83,88.9
N$105  (via drill 1.02)
  other vias: 67.31,88.9
N$106  (via drill 1.02)
  other vias: 62.23,88.9
N$107  (via drill 1.02)
  other vias: 69.85,88.9
N$108  (via drill 1.02)
  other vias: 64.77,88.9
N$109  (via drill 1.02)
  other vias: 72.39,88.9
N$110  (via drill 1.02)
  other vias: 59.69,88.9
N$111  (via drill 1.02)
  other vias: 77.47,86.36
N$112  (via drill 1.02)
  other vias: 57.15,88.9
N$113  (via drill 1.02)
  other vias: 46.99,91.44
N$114  (via drill 1.02)
  other vias: 41.91,91.44
N$115  (via drill 1.02)
  other vias: 49.53,91.44
N$116  (via drill 1.02)
  other vias: 44.45,91.44
N$117  (via drill 1.02)
  other vias: 52.07,91.44
N$118  (via drill 1.02)
  other vias: 39.37,91.44
N$119  (via drill 1.02)
  other vias: 54.61,91.44
N$120  (via drill 1.02)
  other vias: 36.83,91.44
N$121  (via drill 1.02)
  other vias: 67.31,91.44
N$122  (via drill 1.02)
  other vias: 62.23,91.44
N$123  (via drill 1.02)
  other vias: 69.85,91.44
N$124  (via drill 1.02)
  other vias: 64.77,91.44
N$125  (via drill 1.02)
  other vias: 72.39,91.44
N$126  (via drill 1.02)
  other vias: 59.69,91.44
N$127  (via drill 1.02)
  other vias: 74.93,88.9
N$128  (via drill 1.02)
  other vias: 57.15,91.44
N$129  (via drill 1.02)
  other vias: 46.99,93.98
N$130  (via drill 1.02)
  other vias: 41.91,93.98
N$131  (via drill 1.02)
  other vias: 49.53,93.98
N$132  (via drill 1.02)
  other vias: 44.45,93.98
N$133  (via drill 1.02)
  other vias: 52.07,93.98
N$134  (via drill 1.02)
  other vias: 39.37,93.98
N$135  (via drill 1.02)
  other vias: 54.61,93.98
N$136  (via drill 1.02)
  other vias: 36.83,93.98
N$137  (via drill 1.02)
  other vias: 67.31,93.98
N$138  (via drill 1.02)
  other vias: 62.23,93.98
N$139  (via drill 1.02)
  other vias: 69.85,93.98
N$140  (via drill 1.02)
  other vias: 64.77,93.98
N$141  (via drill 1.02)
  other vias: 72.39,93.98
N$142  (via drill 1.02)
  other vias: 59.69,93.98
N$143  (via drill 1.02)
  other vias: 77.47,88.9
N$144  (via drill 1.02)
  other vias: 57.15,93.98
N$145  (via drill 1.02)
  other vias: 46.99,96.52
N$146  (via drill 1.02)
  other vias: 41.91,96.52
N$147  (via drill 1.02)
  other vias: 49.53,96.52
N$148  (via drill 1.02)
  other vias: 44.45,96.52
N$149  (via drill 1.02)
  other vias: 52.07,96.52
N$150  (via drill 1.02)
  other vias: 39.37,96.52
N$151  (via drill 1.02)
  other vias: 54.61,96.52
N$152  (via drill 1.02)
  other vias: 36.83,96.52
N$153  (via drill 1.02)
  other vias: 67.31,96.52
N$154  (via drill 1.02)
  other vias: 62.23,96.52
N$155  (via drill 1.02)
  other vias: 69.85,96.52
N$156  (via drill 1.02)
  other vias: 64.77,96.52
N$157  (via drill 1.02)
  other vias: 72.39,96.52
N$158  (via drill 1.02)
  other vias: 59.69,96.52
N$159  (via drill 1.02)
  other vias: 74.93,91.44
N$160  (via drill 1.02)
  other vias: 57.15,96.52
N$161  (via drill 1.02)
  other vias: 46.99,99.06
N$162  (via drill 1.02)
  other vias: 41.91,99.06
N$163  (via drill 1.02)
  other vias: 49.53,99.06
N$164  (via drill 1.02)
  other vias: 44.45,99.06
N$165  (via drill 1.02)
  other vias: 52.07,99.06
N$166  (via drill 1.02)
  other vias: 39.37,99.06
N$167  (via drill 1.02)
  other vias: 54.61,99.06
N$168  (via drill 1.02)
  other vias: 36.83,99.06
N$169  (via drill 1.02)
  other vias: 67.31,99.06
N$170  (via drill 1.02)
  other vias: 62.23,99.06
N$171  (via drill 1.02)
  other vias: 69.85,99.06
N$172  (via drill 1.02)
  other vias: 64.77,99.06
N$173  (via drill 1.02)
  other vias: 72.39,99.06
N$174  (via drill 1.02)
  other vias: 59.69,99.06
N$175  (via drill 1.02)
  other vias: 77.47,91.44
N$176  (via drill 1.02)
  other vias: 57.15,99.06
N$177  (via drill 1.02)
  other vias: 46.99,101.6
N$178  (via drill 1.02)
  other vias: 41.91,101.6
N$179  (via drill 1.02)
  other vias: 49.53,101.6
N$180  (via drill 1.02)
  other vias: 44.45,101.6
N$181  (via drill 1.02)
  other vias: 52.07,101.6
N$182  (via drill 1.02)
  other vias: 39.37,101.6
N$183  (via drill 1.02)
  other vias: 54.61,101.6
N$184  (via drill 1.02)
  other vias: 36.83,101.6
N$185  (via drill 1.02)
  other vias: 67.31,101.6
N$186  (via drill 1.02)
  other vias: 62.23,101.6
N$187  (via drill 1.02)
  other vias: 69.85,101.6
N$188  (via drill 1.02)
  other vias: 64.77,101.6
N$189  (via drill 1.02)
  other vias: 72.39,101.6
N$190  (via drill 1.02)
  other vias: 59.69,101.6
N$191  (via drill 1.02)
  other vias: 74.93,93.98
N$192  (via drill 1.02)
  other vias: 57.15,101.6
N$193  (via drill 1.02)
  other vias: 46.99,104.14
N$194  (via drill 1.02)
  other vias: 41.91,104.14
N$195  (via drill 1.02)
  other vias: 49.53,104.14
N$196  (via drill 1.02)
  other vias: 44.45,104.14
N$197  (via drill 1.02)
  other vias: 52.07,104.14
N$198  (via drill 1.02)
  other vias: 39.37,104.14
N$199  (via drill 1.02)
  other vias: 54.61,104.14
N$200  (via drill 1.02)
  other vias: 36.83,104.14
N$201  (via drill 1.02)
  other vias: 67.31,104.14
N$202  (via drill 1.02)
  other vias: 62.23,104.14
N$203  (via drill 1.02)
  other vias: 69.85,104.14
N$204  (via drill 1.02)
  other vias: 64.77,104.14
N$205  (via drill 1.02)
  other vias: 72.39,104.14
N$206  (via drill 1.02)
  other vias: 59.69,104.14
N$207  (via drill 1.02)
  other vias: 77.47,93.98
N$208  (via drill 1.02)
  other vias: 57.15,104.14
N$209  (via drill 1.02)
  other vias: 46.99,106.68
N$210  (via drill 1.02)
  other vias: 41.91,106.68
N$211  (via drill 1.02)
  other vias: 49.53,106.68
N$212  (via drill 1.02)
  other vias: 44.45,106.68
N$213  (via drill 1.02)
  other vias: 52.07,106.68
N$214  (via drill 1.02)
  other vias: 39.37,106.68
N$215  (via drill 1.02)
  other vias: 54.61,106.68
N$216  (via drill 1.02)
  other vias: 36.83,106.68
N$217  (via drill 1.02)
  other vias: 67.31,106.68
N$218  (via drill 1.02)
  other vias: 62.23,106.68
N$219  (via drill 1.02)
  other vias: 69.85,106.68
N$220  (via drill 1.02)
  other vias: 64.77,106.68
N$221  (via drill 1.02)
  other vias: 72.39,106.68
N$222  (via drill 1.02)
  other vias: 59.69,106.68
N$223  (via drill 1.02)
  other vias: 74.93,96.52
N$224  (via drill 1.02)
  other vias: 57.15,106.68
N$225  (via drill 1.02)
  other vias: 46.99,109.22
N$226  (via drill 1.02)
  other vias: 41.91,109.22
N$227  (via drill 1.02)
  other vias: 49.53,109.22
N$228  (via drill 1.02)
  other vias: 44.45,109.22
N$229  (via drill 1.02)
  other vias: 52.07,109.22
N$230  (via drill 1.02)
  other vias: 39.37,109.22
N$231  (via drill 1.02)
  other vias: 54.61,109.22
N$232  (via drill 1.02)
  other vias: 36.83,109.22
N$233  (via drill 1.02)
  other vias: 67.31,109.22
N$234  (via drill 1.02)
  other vias: 62.23,109.22
N$235  (via drill 1.02)
  other vias: 69.85,109.22
N$236  (via drill 1.02)
  other vias: 64.77,109.22
N$237  (via drill 1.02)
  other vias: 72.39,109.22
N$238  (via drill 1.02)
  other vias: 59.69,109.22
N$239  (via drill 1.02)
  other vias: 77.47,96.52
N$240  (via drill 1.02)
  other vias: 57.15,109.22
N$241  (via drill 1.02)
  other vias: 46.99,111.76
N$242  (via drill 1.02)
  other vias: 41.91,111.76
N$243  (via drill 1.02)
  other vias: 49.53,111.76
N$244  (via drill 1.02)
  other vias: 44.45,111.76
N$245  (via drill 1.02)
  other vias: 52.07,111.76
N$246  (via drill 1.02)
  other vias: 39.37,111.76
N$247  (via drill 1.02)
  other vias: 54.61,111.76
N$248  (via drill 1.02)
  other vias: 36.83,111.76
N$249  (via drill 1.02)
  other vias: 67.31,111.76
N$250  (via drill 1.02)
  other vias: 62.23,111.76
N$251  (via drill 1.02)
  other vias: 69.85,111.76
N$252  (via drill 1.02)
  other vias: 64.77,111.76
N$253  (via drill 1.02)
  other vias: 72.39,111.76
N$254  (via drill 1.02)
  other vias: 59.69,111.76
N$255  (via drill 1.02)
  other vias: 74.93,99.06
N$256  (via drill 1.02)
  other vias: 57.15,111.76
N$257  (via drill 1.02)
  other vias: 46.99,114.3
N$258  (via drill 1.02)
  other vias: 41.91,114.3
N$259  (via drill 1.02)
  other vias: 49.53,114.3
N$260  (via drill 1.02)
  other vias: 44.45,114.3
N$261  (via drill 1.02)
  other vias: 52.07,114.3
N$262  (via drill 1.02)
  other vias: 39.37,114.3
N$263  (via drill 1.02)
  other vias: 54.61,114.3
N$264  (via drill 1.02)
  other vias: 36.83,114.3
N$265  (via drill 1.02)
  other vias: 67.31,114.3
N$266  (via drill 1.02)
  other vias: 62.23,114.3
N$267  (via drill 1.02)
  other vias: 69.85,114.3
N$268  (via drill 1.02)
  other vias: 64.77,114.3
N$269  (via drill 1.02)
  other vias: 72.39,114.3
N$270  (via drill 1.02)
  other vias: 59.69,114.3
N$271  (via drill 1.02)
  other vias: 77.47,99.06
N$272  (via drill 1.02)
  other vias: 57.15,114.3
N$273  (via drill 1.02)
  other vias: 46.99,116.84
N$274  (via drill 1.02)
  other vias: 41.91,116.84
N$275  (via drill 1.02)
  other vias: 49.53,116.84
N$276  (via drill 1.02)
  other vias: 44.45,116.84
N$277  (via drill 1.02)
  other vias: 52.07,116.84
N$278  (via drill 1.02)
  other vias: 39.37,116.84
N$279  (via drill 1.02)
  other vias: 54.61,116.84
N$280  (via drill 1.02)
  other vias: 36.83,116.84
N$281  (via drill 1.02)
  other vias: 67.31,116.84
N$282  (via drill 1.02)
  other vias: 62.23,116.84
N$283  (via drill 1.02)
  other vias: 69.85,116.84
N$284  (via drill 1.02)
  other vias: 64.77,116.84
N$285  (via drill 1.02)
  other vias: 72.39,116.84
N$286  (via drill 1.02)
  other vias: 59.69,116.84
N$287  (via drill 1.02)
  other vias: 74.93,101.6
N$288  (via drill 1.02)
  other vias: 57.15,116.84
N$289  (via drill 1.02)
  other vias: 46.99,119.38
N$290  (via drill 1.02)
  other vias: 41.91,119.38
N$291  (via drill 1.02)
  other vias: 49.53,119.38
N$292  (via drill 1.02)
  other vias: 44.45,119.38
N$293  (via drill 1.02)
  other vias: 52.07,119.38
N$294  (via drill 1.02)
  other vias: 39.37,119.38
N$295  (via drill 1.02)
  other vias: 54.61,119.38
N$296  (via drill 1.02)
  other vias: 36.83,119.38
N$297  (via drill 1.02)
  other vias: 67.31,119.38
N$298  (via drill 1.02)
  other vias: 62.23,119.38
N$299  (via drill 1.02)
  other vias: 69.85,119.38
N$300  (via drill 1.02)
  other vias: 64.77,119.38
N$301  (via drill 1.02)
  other vias: 72.39,119.38
N$302  (via drill 1.02)
  other vias: 59.69,119.38
N$303  (via drill 1.02)
  other vias: 77.47,101.6
N$304  (via drill 1.02)
  other vias: 57.15,119.38
N$305  (via drill 1.02)
  other vias: 90.17,104.14
N$306  (via drill 1.02)
  other vias: 85.09,104.14
N$307  (via drill 1.02)
  other vias: 92.71,104.14
N$308  (via drill 1.02)
  other vias: 87.63,104.14
N$309  (via drill 1.02)
  other vias: 95.25,104.14
N$310  (via drill 1.02)
  other vias: 82.55,104.14
N$311  (via drill 1.02)
  other vias: 74.93,104.14
N$312  (via drill 1.02)
  other vias: 80.01,104.14
N$313  (via drill 1.02)
  other vias: 90.17,106.68
N$314  (via drill 1.02)
  other vias: 85.09,106.68
N$315  (via drill 1.02)
  other vias: 92.71,106.68
N$316  (via drill 1.02)
  other vias: 87.63,106.68
N$317  (via drill 1.02)
  other vias: 95.25,106.68
N$318  (via drill 1.02)
  other vias: 82.55,106.68
N$319  (via drill 1.02)
  other vias: 77.47,104.14
N$320  (via drill 1.02)
  other vias: 80.01,106.68
N$321  (via drill 1.02)
  other vias: 90.17,109.22
N$322  (via drill 1.02)
  other vias: 85.09,109.22
N$323  (via drill 1.02)
  other vias: 92.71,109.22
N$324  (via drill 1.02)
  other vias: 87.63,109.22
N$325  (via drill 1.02)
  other vias: 95.25,109.22
N$326  (via drill 1.02)
  other vias: 82.55,109.22
N$327  (via drill 1.02)
  other vias: 74.93,106.68
N$328  (via drill 1.02)
  other vias: 80.01,109.22
N$329  (via drill 1.02)
  other vias: 90.17,111.76
N$330  (via drill 1.02)
  other vias: 85.09,111.76
N$331  (via drill 1.02)
  other vias: 92.71,111.76
N$332  (via drill 1.02)
  other vias: 87.63,111.76
N$333  (via drill 1.02)
  other vias: 95.25,111.76
N$334  (via drill 1.02)
  other vias: 82.55,111.76
N$335  (via drill 1.02)
  other vias: 77.47,106.68
N$336  (via drill 1.02)
  other vias: 80.01,111.76
N$337  (via drill 1.02)
  other vias: 90.17,114.3
N$338  (via drill 1.02)
  other vias: 85.09,114.3
N$339  (via drill 1.02)
  other vias: 92.71,114.3
N$340  (via drill 1.02)
  other vias: 87.63,114.3
N$341  (via drill 1.02)
  other vias: 95.25,114.3
N$342  (via drill 1.02)
  other vias: 82.55,114.3
N$343  (via drill 1.02)
  other vias: 74.93,109.22
N$344  (via drill 1.02)
  other vias: 80.01,114.3
N$345  (via drill 1.02)
  other vias: 90.17,116.84
N$346  (via drill 1.02)
  other vias: 85.09,116.84
N$347  (via drill 1.02)
  other vias: 92.71,116.84
N$348  (via drill 1.02)
  other vias: 87.63,116.84
N$349  (via drill 1.02)
  other vias: 95.25,116.84
N$350  (via drill 1.02)
  other vias: 82.55,116.84
N$351  (via drill 1.02)
  other vias: 77.47,109.22
N$352  (via drill 1.02)
  other vias: 80.01,116.84
N$353  (via drill 1.02)
  other vias: 90.17,119.38
N$354  (via drill 1.02)
  other vias: 85.09,119.38
N$355  (via drill 1.02)
  other vias: 92.71,119.38
N$356  (via drill 1.02)
  other vias: 87.63,119.38
N$357  (via drill 1.02)
  other vias: 95.25,119.38
N$358  (via drill 1.02)
  other vias: 82.55,119.38
N$359  (via drill 1.02)
  other vias: 74.93,111.76
N$360  (via drill 1.02)
  other vias: 80.01,119.38
N$361  (via drill 1.02)
  other vias: 77.47,111.76
N$362  (via drill 1.02)
  other vias: 74.93,114.3
N$363  (via drill 1.02)
  other vias: 77.47,114.3
N$364  (via drill 1.02)
  other vias: 74.93,116.84
N$365  (via drill 1.02)
  other vias: 77.47,116.84
N$366  (via drill 1.02)
  other vias: 74.93,119.38
N$367  (via drill 1.02)
  other vias: 77.47,119.38
PE  (via drill 0.3 pad 0.61)
  Top 0.406: v1.43,76.2 USB1.M2 | USB1.M1 v1.43,65.72
  Bottom 1.016: XT-NANO-SXL.SHIELD 34,7.7 34.24,7.46
  pour Bottom: 0.5,1.5 1.5,0.5 98.5,0.5 99.5,1.5 99.5,7.5 98.5,8.5 70,8.5 69,7.5 69,5.5 67.5,3.5 60,3.5 58,5.5 58,7.5 57,8.5 27.5,8.5 26.5,7.5 26.5,5.5 24.5,3.5 17.5,3.5 15.5,5.5 15.5,7.5 14.5,8.5 3.5,8.5 2.5,9.5 2.5,77.34 10.16,77.34 11.16,78.34 11.16,80.5 10.16,81.5 2.5,81.5 2.5,89.5 3.5,90.5 10.16,90.5 11.16,91.5 11.16,93.66 10.16,94.66 2.5,94.66 2.5,97.5 11.5,97.5 12.5,98.5 12.5,102.5 11.5,103.5 6,103.5 4.5,105 4.5,121.5 5.5,122.5 11.5,122.5 12.5,123.5 12.5,127.5 11.5,128.5 4.5,128.5 3.5,129.5 3.5,159.5 0.5,159.5
PGEC2
  Top 0.203: ISP.5 83.03,14.58 83.03,15.24 68.45,29.82 51.59,29.84 51.45,29.84 ISP1.2 50.69,30.59
  Bottom 0.203: ISP3.2 25,60.56 26.04,61.59 32.38,61.59 33.66,60.33 33.66,42.55 33.97,42.23 49.05,42.23 52.55,38.73 52.55,32.47 ISP1.2 50.82,30.48 55.56,30.48 66.69,41.61 ISP2.2
PGED2
  Top 0.203: ISP.4 81.76,12.04 81.76,15.88 68.26,29.37 51.59,29.37 50.84,28.61 ISP1.1
  Bottom 0.203: ISP3.1 27,60.02 27.94,60.96 32.23,60.96 33.18,60.01 33.18,42.23 33.66,41.75 48.9,41.75 52.07,38.58 52.07,33.97 49.21,31.11 49.21,28.89 49.53,28.57 50.66,28.57 ISP1.1 50.73,28.57 54.77,28.57 65.8,39.61 ISP2.1
POE12  (via drill 0.3 pad 0.61)
  Top 0.406: XT-PICO-SXL.P3_7 67.5,22.76 63.91,26.35 v34.08,26.35 32.18,26.35 27.26,21.43 v24.13,21.43 | T2.15 24.18,18.05 v24.13,18.1
  Bottom 0.406: v34.08,26.35 34.08,17.08 XT-NANO-SXL.POE12 | v24.13,18.1 v24.13,21.43 | XT-PICO-SXL.P3_7 67.5,22.76 68.71,23.97 78.58,23.97 83.45,19.1 POWER_OVER_ETHERNET-MODUL.1
POE36  (via drill 0.3 pad 0.61)
  Top 0.406: XT-PICO-SXL.P3_6 65.5,22.85 62.79,25.56 v49.96,25.56 32.5,25.56 27.57,20.64 18.26,20.64 17.82,20.21 T2.10
  Bottom 0.406: v49.96,25.56 49.96,17.12 XT-NANO-SXL.POE36 | XT-PICO-SXL.P3_6 65.48,22.09 65.48,23.18 67.07,24.77 79.14,24.77 82.26,21.64 POWER_OVER_ETHERNET-MODUL.2
POE45  (via drill 0.3 pad 0.61)
  Top 0.406: XT-PICO-SXL.P3_5 63.5,22.95 61.68,24.77 v46.35,24.77 40.59,24.77 35.67,19.84 v30.32,19.84
  Bottom 0.406: RJ1.5 21.51,6.56 RJ1.4 21.51,9.13 22.07,9.68 29.53,9.68 30.32,10.48 v30.32,19.84 | XT-PICO-SXL.P3_5 63.34,22.16 63.34,23.18 65.72,25.56 79.69,25.56 81.12,24.13 89.02,24.13 POWER_OVER_ETHERNET-MODUL.3 | XT-NANO-SXL.POE45 47.39,15 46.35,16.03 v46.35,24.77
POE78  (via drill 0.3 pad 0.61)
  Top 0.406: XT-PICO-SXL.P3_4 61.5,23.04 60.57,23.97 40.96,23.97 v37.94,20.95 36.04,19.05 v29.37,19.05
  Bottom 0.406: RJ1.7 17.44,6.56 RJ1.8 17.44,8.71 19.37,10.64 28.89,10.64 29.37,11.11 v29.37,19.05 | XT-PICO-SXL.P3_4 61.44,22.06 61.44,23.18 64.58,26.32 88.67,26.32 POWER_OVER_ETHERNET-MODUL.4 | v37.94,20.95 37.94,16.19 36.75,15 XT-NANO-SXL.POE78
RD+  (via drill 0.3 pad 0.61)
  Top 0.203: T2.6 19.09,23.85 v19.13,23.81
  Top 0.305: T2.6 19.09,26.56 19.37,26.83 R4.1 | M1.P2_6 XT-FEMTO-SXL.P2_6
  Bottom 0.203: XT-FEMTO-SXL.P2_6 23.16,36.02 24.29,36.04 24.45,36.04 27.3,33.18 27.3,24.29 26.35,23.18 19.37,23.18 19.13,23.42 v19.13,23.81
RD-  (via drill 0.3 pad 0.61)
  Top 0.203: T2.8 16.55,23.86 v16.51,23.81
  Top 0.305: T2.8 16.55,26.47 16.19,26.83 R5.1 | M1.P2_5 XT-FEMTO-SXL.P2_5
  Bottom 0.203: XT-FEMTO-SXL.P2_5 21,36.56 21.59,37.15 23.97,37.15 27.78,33.34 27.78,24.13 26.51,22.7 16.99,22.7 16.51,23.18 v16.51,23.81
RS232_CTS_A  (via drill 0.3 pad 0.61)
  Top 0.203: v16.83,113.51 15.45,113.51 U4.6
  Bottom 0.203: RS232.8 12.28,111.66 14.13,113.51 v16.83,113.51
RS232_DCD_A
  Top 0.203: RS232.1 14.04,114.87 14.04,114.83 U4.4
RS232_DSR_A
  Top 0.203: RS232.6 11.12,117.14 14.05,114.22 14.05,114.18 U4.5
RS232_DTR_A
  Top 0.203: 10.41,110.32 RS232.4 10.38,110.28 U4.11
RS232_RI_A  (via drill 0.3 pad 0.61)
  Top 0.203: U4.8 14.29,112.23 v14.29,112.24
  Bottom 0.203: v14.29,112.24 10.95,108.9 7.85,108.9 RS232.9
RS232_RTS_A
  Top 0.203: RS232.7 7.94,114.3 11.27,114.3 13.95,111.62 13.95,111.58 U4.9
RS232_RXD_A
  Top 0.203: RS232.2 11.23,115.77 14.08,112.92 14.08,112.88 U4.7
RS232_TXD_A
  Top 0.203: RS232.3 12.44,110.97 12.44,110.93 U4.10
RS485_A
  Top 0.203: R2U6.2 R3U6.2 82.55,147 83.19,146.37 U6.6 91.92,146.37 93.03,145.26 93.03,139.86 92.08,138.91 RS485.2
RS485_B
  Top 0.203: RS485.1 92.39,133.83 94.3,135.73 94.3,145.73 92.39,147.64 U6.7 83.5,147.64 83.19,147.96 83.19,149.86 83.82,150.5 83.82,150.97 | JP1.5 80.17,156.69 81.44,155.42 83.19,155.42 83.82,154.78 83.82,150.97 | R1U6.2 83.89,150.9 83.82,150.97
RX+
  Top 0.203: T2.11 19.09,13.29 22.54,9.84 22.54,5.56 RJ1.3
RX-
  Top 0.203: T2.9 16.55,14.56 19.37,11.75 19.37,7.43 RJ1.6
SD_SPI_CLK
  Top 0.203: SD1.5 11.35,142.32 13.02,140.65 16.51,140.65 P2.3
SD_SPI_CS
  Top 0.203: SD1.2 11.16,139.02 14.13,136.05 P2.4
SD_SPI_MISO
  Top 0.203: SD1.7 9.95,144.52 13.34,141.13 P2.2
SD_SPI_MOSI
  Top 0.203: SD1.3 10.85,140.12 13.65,137.32 20.8,137.32 21.11,137.64 21.11,143.03 20.48,143.67 P2.1
TD+  (via drill 0.3 pad 0.61)
  Top 0.203: T2.1 25.45,23.85 v25.48,23.81
  Top 0.305: T2.1 25.45,26.56 25.72,26.83 R10.1 | M1.P2_4 XT-FEMTO-SXL.P2_4
  Bottom 0.203: XT-FEMTO-SXL.P2_4 19,35.29 20.16,34.13 25.72,34.13 26.83,33.02 26.83,24.45 26.19,23.81 v25.48,23.81
TD-  (via drill 0.3 pad 0.61)
  Top 0.203: T2.3 22.91,23.86 v22.86,23.81
  Top 0.305: T2.3 22.91,26.47 22.54,26.83 R8.1 | M1.P2_3 XT-FEMTO-SXL.P2_3
  Bottom 0.203: XT-FEMTO-SXL.P2_3 17,34.91 18.26,33.66 25.56,33.66 26.35,32.86 26.35,24.77 26.19,24.61 23.65,24.61 v22.86,23.81
TTL485_!R!/W
  Top 0.203: U6.3 81.12,146.37 | 81.12,146.37 81.44,146.05 81.44,144.62 80.49,143.67 80.49,141.29 80.8,140.97 84.14,140.97 84.61,140.49 84.61,134.94 84.3,134.62 P4.4 | U6.2 80.96,147.64 81.12,147.48 81.12,146.37
TTL485_RXD
  Top 0.203: U6.1 81.12,148.91 81.76,148.27 81.76,146.69 82.55,145.89 P4.1
TTL485_TXD
  Top 0.203: U6.4 79.33,140.54 80.17,139.7 P4.2
TTL_CTS0
  Top 0.152: XT-PICO-SXL.P1_4 61.5,42.13 60.96,41.59 44.45,41.59 40.96,38.1 40.96,35.96 XT-NANO-SXL.P1_4
  Top 0.203: M1.P1_3 XT-FEMTO-SXL.P1_3
  Bottom 0.152: XT-NANO-SXL.P1_4 40.96,35.96 40.96,37.94 39.37,39.53 27.94,39.53 26.67,40.8 26.67,50.32 27.3,50.96 30.96,50.96 31.59,50.32 31.59,48.74 30.86,48 XT-FEMTO-SXL.P1_3 | PORT1.6 41.91,67.63 60.48,49.05 60.48,47.02 XT-PICO-SXL.P1_4
TTL_CTS1  (via drill 0.3 pad 0.61)
  Top 0.152: XT-NANO-SXL.P2_4 40.01,38.1 43.81,41.91 60.01,41.91 60.48,42.39 60.48,46.83 61.5,47.85 XT-PICO-SXL.P2_4 61.5,78.01 PORT2.6 | XT-NANO-SXL.P2_4 | XT-NANO-SXL.P2_4 40.01,36.51 39.05,35.56 39.05,32.54 v38.89,32.38
  Top 0.203: M1.P3_3 XT-FEMTO-SXL.P3_3
  Bottom 0.152: XT-FEMTO-SXL.P3_3 17.09,48 32.38,32.7 38.58,32.7 v38.89,32.38
TTL_CTS_A
  Top 0.203: U4.17 25.15,109.63 26.19,108.58 P1.6
TTL_DCD0
  Top 0.152: XT-PICO-SXL.P2_1 55.46,48 54.45,46.99 54.45,43.81 53.82,43.18 41.12,43.18 36.04,38.1 35.1,38.1 XT-NANO-SXL.P2_1 33.99,36.99 31.91,36.99 30.7,38.2 M1.P1_6
  Top 0.203: XT-FEMTO-SXL.P1_6 M1.P1_6
  Bottom 0.152: PORT1.7 39.37,65.25 55.56,49.05 55.56,48.06 XT-PICO-SXL.P2_1
TTL_DCD1  (via drill 0.3 pad 0.61)
  Top 0.152: v36.99,31.43 36.99,35.88 38,36.89 XT-NANO-SXL.P2_3 38,37.84 42.7,42.55 57.94,42.55 58.5,43.1 58.5,46.91 59.5,47.91 XT-PICO-SXL.P2_3 59.5,78.55 PORT2.7
  Top 0.203: M1.P3_6 XT-FEMTO-SXL.P3_6 | JMP1.3 51.23,48.69 v51.28,48.74
  Route15 0.203: v51.28,48.74 53.18,48.74 54.13,49.69 57.81,49.69 XT-PICO-SXL.P2_3
  Bottom 0.152: XT-FEMTO-SXL.P3_6 21.66,42 31.91,31.75 36.67,31.75 v36.99,31.43
TTL_DCD_A
  Top 0.203: U4.19 24.64,110.93 25.72,109.86 29.69,109.86 30.32,109.22 30.32,106.52 29.84,106.05 P1.7
TTL_DSR0
  Top 0.152: XT-PICO-SXL.P1_7 67.5,42.89 64.29,39.69 48.74,39.69 46.99,37.94 46.99,35.99 XT-NANO-SXL.P1_7
  Top 0.203: XT-FEMTO-SXL.P1_5 M1.P1_5
  Bottom 0.152: XT-NANO-SXL.P1_7 46.99,35.99 46.99,37.94 44.45,40.48 28.42,40.48 27.62,41.27 27.62,43.66 27.94,43.97 28.97,43.97 XT-FEMTO-SXL.P1_5 | PORT1.3 49.53,66.04 66.52,49.05 66.52,46.98 XT-PICO-SXL.P1_7
TTL_DSR1
  Top 0.152: XT-NANO-SXL.P2_7 46.04,37.04 46.04,37.94 48.1,40.01 64.14,40.01 66.52,42.39 66.52,46.99 67.5,47.97 XT-PICO-SXL.P2_7 67.5,76.39 PORT2.3
  Top 0.203: M1.P3_5 XT-FEMTO-SXL.P3_5
  Bottom 0.152: XT-FEMTO-SXL.P3_5 20.14,44 32.07,32.07 37.94,32.07 38.58,31.43 43.81,31.43 45.01,32.62 45.01,35.56 46,36.55 XT-NANO-SXL.P2_7
TTL_DSR_A
  Top 0.203: U4.18 21.64,110.28 20.64,111.28 20.64,116.84 21.59,117.79 26.67,117.79 P1.3
TTL_DTR0
  Top 0.152: XT-PICO-SXL.P1_6 65.5,41.85 63.98,40.32 47.47,40.32 45.01,37.86 45.01,36.01 XT-NANO-SXL.P1_6
  Top 0.203: XT-FEMTO-SXL.P1_4 M1.P1_4
  Bottom 0.152: XT-FEMTO-SXL.P1_4 28.96,46.04 27.62,46.04 27.3,45.72 27.3,41.12 28.26,40.16 42.7,40.16 45.01,37.86 45.01,36.01 XT-NANO-SXL.P1_6 | PORT1.4 46.99,66.52 64.53,48.97 64.53,46.97 XT-PICO-SXL.P1_6
TTL_DTR1
  Top 0.152: XT-NANO-SXL.P2_6 43.97,37.03 43.97,37.94 46.67,40.64 63.82,40.64 64.45,41.27 64.45,46.99 65.46,48 XT-PICO-SXL.P2_6 65.5,76.93 PORT2.4
  Top 0.203: M1.P3_4 XT-FEMTO-SXL.P3_4
  Bottom 0.152: XT-FEMTO-SXL.P3_4 18.61,46 32.23,32.38 38.1,32.38 38.73,31.75 41.75,31.75 43.02,33.02 43.02,35.56 43.97,36.51 43.97,36.97 XT-NANO-SXL.P2_6
TTL_DTR_A
  Top 0.203: U4.12 18.51,109.63 19.37,110.49 19.37,118.59 23.81,123.03 30,123.03 30.8,122.24 30.8,114.3 30.16,113.67 P1.4
TTL_RI1
  Top 0.152: XT-NANO-SXL.P2_2 37.1,38.1 37.15,38.1 41.91,42.86 55.72,42.86 56.52,43.66 56.52,46.99 57.5,47.98 XT-PICO-SXL.P2_2 57.5,79.09 PORT2.8
TTL_RI_A
  Top 0.203: U4.15 25.34,108.33 26.19,107.47 26.19,103.98 26.67,103.5 P1.8
TTL_RTS0
  Top 0.152: XT-PICO-SXL.P1_5 63.5,41.59 62.87,40.96 45.88,40.96 43.02,38.1 43.02,36.02 XT-NANO-SXL.P1_5
  Top 0.203: XT-FEMTO-SXL.P1_2 M1.P1_2
  Bottom 0.152: XT-NANO-SXL.P1_5 43.02,36.02 43.02,38.1 41.27,39.85 28.1,39.85 26.99,40.96 26.99,49.53 27.46,50.01 XT-FEMTO-SXL.P1_2 | PORT1.5 44.45,66.99 62.55,48.9 62.55,46.95 XT-PICO-SXL.P1_5
TTL_RTS1
  Top 0.152: XT-NANO-SXL.P2_5 42,38.03 45.24,41.27 61.91,41.27 62.55,41.91 62.55,46.99 63.5,47.94 XT-PICO-SXL.P2_5 63.5,77.47 PORT2.5
  Top 0.203: M1.P3_2 XT-FEMTO-SXL.P3_2
  Bottom 0.152: XT-FEMTO-SXL.P3_2 15.56,50 32.54,33.02 39.05,33.02 39.69,32.38 40.32,32.38 41.04,33.1 41.04,35.56 42,36.52 XT-NANO-SXL.P2_5
TTL_RTS_A
  Top 0.203: U4.14 20.58,108.33 21.27,107.63 24.92,107.63 25.72,106.84 25.72,103.03 26.67,102.08 29.84,102.08 30.8,103.03 30.8,110.65 30.32,111.12 P1.5
TTL_RXD0
  Top 0.152: XT-PICO-SXL.P1_9 71.5,44.99 64.93,38.42 53.42,38.42 XT-NANO-SXL.P1_9
  Top 0.203: XT-FEMTO-SXL.P1_1 M1.P1_1
  Bottom 0.152: XT-NANO-SXL.P1_9 51.12,36.12 51.12,37.94 47.94,41.12 33.02,41.12 32.54,41.59 32.54,54.29 31.75,55.09 28.1,55.09 27.78,54.77 27.78,52.86 28.64,52 XT-FEMTO-SXL.P1_1 | PORT1.1 54.61,64.93 70.48,49.05 70.48,47.02 XT-PICO-SXL.P1_9
TTL_RXD1  (via drill 0.3 pad 0.61)
  Top 0.152: v39.85,33.02 48.26,33.02 49.05,33.81 49.05,35.56 50,36.51 XT-NANO-SXL.P2_9 51.73,38.73 64.77,38.73 70.48,44.45 70.48,46.99 XT-PICO-SXL.P2_9 71.5,75.31 PORT2.1
  Top 0.203: M1.P3_1 XT-FEMTO-SXL.P3_1
  Bottom 0.152: XT-FEMTO-SXL.P3_1 14.04,52 32.7,33.34 39.53,33.34 v39.85,33.02
TTL_RXD_A
  Top 0.203: U4.16 21.51,108.98 20.24,110.25 20.24,118.19 23.34,121.28 P1.1
TTL_TXD0
  Top 0.152: XT-PICO-SXL.P1_8 69.5,43.94 64.61,39.05 50.01,39.05 49.05,38.1 49.05,36.05 XT-NANO-SXL.P1_8
  Top 0.203: XT-FEMTO-SXL.P1_0 M1.P1_0
  Bottom 0.152: XT-NANO-SXL.P1_8 49.05,36.05 49.05,37.78 46.04,40.8 32.7,40.8 32.23,41.27 32.23,53.02 31.27,53.98 29.02,53.98 XT-FEMTO-SXL.P1_0 | PORT1.2 52.07,65.41 68.5,48.97 68.5,47 XT-PICO-SXL.P1_8
TTL_TXD1  (via drill 0.3 pad 0.61)
  Top 0.152: v40.32,33.66 46.67,33.66 46.99,33.97 46.99,35.48 48,36.49 XT-NANO-SXL.P2_8 48,37.84 49.53,39.37 64.45,39.37 68.5,43.42 68.5,46.91 69.5,47.91 XT-PICO-SXL.P2_8 69.5,75.85 PORT2.2
  Top 0.203: M1.P3_0 XT-FEMTO-SXL.P3_0
  Bottom 0.152: XT-FEMTO-SXL.P3_0 12.52,54 32.86,33.66 v40.32,33.66
TTL_TXD_A
  Top 0.203: U4.13 18.65,108.98 19.84,110.17 19.84,118.43 23.97,122.56 29.69,122.56 30.32,121.92 30.32,119.06 30,118.75 P1.2
TX+
  Top 0.203: T2.16 25.45,15.13 24.29,13.97 24.29,9.05 25.08,8.26 25.08,6.07 RJ1.1
TX-
  Top 0.203: RJ1.2 23.54,13.77 23.42,13.89 23.02,14.29 22.91,14.4 T2.14
USB_DM
  Top 0.203: XT-FEMTO-SXL.P4_2 M1.P4_2 15,70.09 13.34,71.75 11.85,71.75 L1U5.1
USB_DP
  Top 0.203: XT-FEMTO-SXL.P4_1 M1.P4_1 13,69.71 11.91,70.8 11.22,70.8 L1U5.4
USB_ID
  Top 0.203: XT-FEMTO-SXL.P4_0 M1.P4_0 11,68.53 9.53,70.01 6.19,70.01 5.89,70.31 USB1.4
  Bottom 0.305: JPU5.2 12.43,69.85 11,68.42 XT-FEMTO-SXL.P4_0
V-POE
  Top 0.813: JX1.2 88.5,79.77 85.57,76.83 CP4.+ 85.41,75.49 83.5,73.66 RB1.1 89.05,64.84 POWER_OVER_ETHERNET-MODUL.8
VBUS
  Top 0.203: M1.P4_3 XT-FEMTO-SXL.P4_3
  Top 0.305: L2U5.1 18.79,90.99 C3U5.2 | U5.1 23.71,79.09 24.29,78.51 24.29,65.56 23.18,64.45 17.62,64.45 17,63.83 M1.P4_3 | RD3.1 D1U5.A
  Top 0.406: L2U5.1 21.43,89.53 22.7,88.27 22.7,88.26 C2U5.+ | D1U5.A 27.93,83.8 C2U5.+ | C2U5.+ U5.1

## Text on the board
Top: RoHS | EVA-KIT-30052015
Bottom: RoHS
tNames: SD-CARD | GND | MOSI | RXD | MISO | TXD | A | SCK | !CS | !R!/W | B | SPI | RS485 | SPI | +3.3 Volt | GND | !RS | !CS | SCK | MISO | MOSI | RXD | TXD | DSR | DTR | RTS | CTS | DCD | RI | RS232 | +5 Volt | PORT1 | PORT2 | RS232 | RS232 | NC | DCD | CTS | RTS | DTR | DSR | TXD | RXD | RI | DCD | CTS | RTS | DTR | DSR | TXD | RXD | RS485 | RS485 | !R!/W | TXD | RXD | !R!/W | TXD | RXD | !RS | !CS | SCK | MISO | MOSI | SPI | !RS | !CS | SCK | MISO | MOSI | SPI | SDA | SCL | I2C | SDA | SCL | I2C | PIN7 | PIN4 | PIN3 | PIN5 | PIN6 | PIN1 | PIN2 | TTLIO | PIN8 | PIN7 | PIN4 | PIN3 | PIN5 | PIN6 | PIN1 | PIN2 | TTLIO
Bemassung: 160.00 | 0.00 | 0.00 | 100.00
